(* Logix 5000 AddOnInstructionDefinition export Banner_Q5X_2000_Param_v4; software revision 33.00 *)

TYPE Banner_IOL_Port_v4 :   // UDT that has all of the data items necessary to communicate with a specific Port on a IO-Link Master
STRUCT
   Port_Controlled : INT;   // Each bit represents a port on an IO-Link Master. Set to 1 to tell AOI to control that port.
   Port_Activate : INT;   // Each bit represents a port on an IO-Link Master. When ON that port will process any commands in queue.
   Port_Read : INT;   // Each bit represents a port on an IO-Link Master. Used to determine when device AOI has requested a Read command.
   Port_Write : INT;   // Each bit represents a port on an IO-Link Master. Used to determine when device AOI has requested a Write command.
   Port_RW_Complete : INT;   // Each bit represents a port on an IO-Link Master. Tells device AOI that Read or Write request has been completed.
   Port_Device_Read : INT;
   Data_Transfer : SINT[190];   // Array to transfer data from IO-Master to device AOIs.
END_STRUCT
END_TYPE

TYPE Banner_Q5X_2000_RD_v4 :   // UDT that stores the Write Data for a Q5X.
STRUCT
   Master_Cycle_Time : INT;
   Min_Cycle_Time : INT;
   M_Sequence_Capability : INT;
   IO_Link_Version_ID : INT;
   Process_Data_Input_Length : INT;
   Process_Data_Output_Length : INT;
   Combined_Vendor_ID : DINT;   // IO-Link Vendor ID
   Vendor_ID1 : INT;
   Vendor_ID2 : INT;
   Combined_Device_ID : DINT;   // IO-Link Device ID
   Device_ID1 : INT;
   Device_ID2 : INT;
   Device_ID3 : INT;
   Serial_Number : STRING;
   Teach_State : SINT;   // 0 =IDLE, 1 = SP1 Success, 4 = Wait for Command, 5 = Busy, 7 = Error
   SP1_TP1 : SINT;   // 0 = not taught or unsuccessful, 1 = successfully taught
   SP2_TP2 : SINT;   // 0 = not taught or unsuccessful, 1 = successfully taught
   Measurement_Value : DINT;   // Measurement value in .1 mm. Dual mode the value is in percent match to taught object.
   Excess_Gain_Percent : DINT;   // Excess gain expressed as a percentage of minimum signal strength.
   Stability : INT;   // 0 = No target exists, 1 = Marginal or multiple peaks, 2 = Stable
   Multiple_Peak_State : INT;   // 0 = Multiple peaks not present, 1 = Multiple peaks present
   Emitter_Status : INT;   // 0 = Active 1 = Inactive.
   Laser_Fault_Status : INT;   // 0 = Not present, 1 Laser fault present
   BDC1_Totalizer_Counts : DINT;   // Number of totalizer edges seen on BDC1. Range: 0 to 65535.
   BDC2_Totalizer_Counts : DINT;   // Number of totalizer edges seen on BDC2. Range: 0 to 65535.
   All_Time_Run_Time : DINT;   // 0 to 2 Million. 1/4 hr increments.
   Display_String : STRING;   // String currently being displayed on the LED display of the sensor
END_STRUCT
END_TYPE

TYPE Banner_Q5X_2000_v4 :   // All of the parameters for a Q5X.
STRUCT
   Initial_Global_Read : BOOL;   // Determines if all of the IO-Link data has been read into the PLC yet
   Command : INT;   // Value placed in here will activate a read or write to a specifc IO-Link Index
   Read : Banner_Q5X_2000_RD_v4;   // Read Only Data
   Write : Banner_Q5X_2000_WD_v4;   // Write Data
   Archive_Data : Banner_Q5X_2000_WD_v4;   // Archive Write Data
   Reset : BOOL;   // Resets AOI. This will force a complete parameter read of the sensor.
END_STRUCT
END_TYPE

TYPE Banner_Q5X_2000_WD_v4 :   // UDT that stores the Write Data for a Q5X.
STRUCT
   System_Command : INT;   // See IODD file for list of commands that can be activated via the System Command interface
   Parameter_Access_Lock : SINT;   // Write access to all parameters is prohibited while value is 1. Only this parameter can be adjusted when value is 1.
   Data_Storage_Lock : SINT;   // Automatic data storage is disabled when this value is equal to 1. Read access is not affected.
   Local_Parameterization_Lock : SINT;   // Parameterization via local control elements on device is disabled.
   Local_User_Interface_Lock : SINT;   // Operation of local user interface is disabled.
   Teach_Channel : INT;   // 0 = Default, 1 = BDC1, 2 = BDC2
   BDC1_Setpoint_SP1 : DINT;   // Switch point value in .1 mm increments. Range: varies depending on sensor.
   BDC1_Setpoint_SP2 : DINT;   // In FGS mode defines second switching point parameter. Range: varies depending on sensor.
   BDC1_Swithpoint_Logic : INT;   // 0 = Light Operate, 1 = Dark Operate
   BDC1_BDC_Mode : INT;   // 1 = 1-Pt BGS, 128 = 2-Pt, 129 = Dynamic, 130 = Window or FGS, 131 = Dual
   BDC1_Hysteresis : DINT;   // Should always be 0
   BDC2_Setpoint_SP1 : DINT;   // Switch point value in .1 mm increments. Range: varies depending on sensor.
   BDC2_Setpoint_SP2 : DINT;   // In FGS mode defines second switching point parameter. Range: varies depending on sensor.
   BDC2_Switchpoint_Logic : INT;   // 0 = Light Operate, 1 = Dark Operate
   BDC2_BDC_Mode : INT;   // 1 = 1-Pt BGS, 128 = 2-Pt, 129 = Dynamic, 130 = Window or FGS, 131 = Dual
   BDC2_Hysteresis : DINT;   // Should always be 0
   Response_Speed : INT;   // 0 = 1.5 ms, 1 = 3 ms, 2 = 10 ms, 3 = 25 ms, 4 = 50 ms
   Gain : INT;   // 0 = High excess gain mode, 1 = Standard excess gain mode
   Secondary_Output_Function : INT;   // 0 = Independent Output, 1 = Complimentary Output, 2 = Remote Teach Input, 3 = Laser Off, 4 = Laser On, 5 = Master, 6 = Slave, 7 = Pulse Frequency Modulation
   Zero_Reference_Location : INT;   // 0 = Near, 1 = Far
   Shift_Zero_Reference_After_Teach : INT;   // 0 = On, 1 = Off
   Display_Read : INT;   // 0 = On, 1 = On Inverted, 2 Off, 3 Off Inverted
   Pushbutton_Lockout : INT;   // 0 = No lockout, 1 = Pushbuttons locked, 2 = Operator Lockout
   Output_Polarity : INT;   // 0 = Default, 1 = PNP, 2 = NPN.
   IOL_Filter_Time : DINT;   // Time to average IOL process data measurement between updates. Range 0 to 65535 ms.
   Include_Binary_Data : INT;   // 0 = Include, 1 = Don't Include.
   Measurement_1_Selection : INT;   // 0 = Disabled, 1 = Excess Gain, 2 = Excess Gain/10, 3 = Channel 1 Dual Mode Percent
   Measurement_2_Selection : INT;   // 0 = Disabled, 1 = Distance Measurement (divide by 10 to get cm value), 2 = Displayed Measurment, 3 = Channel 2 Dual Mode Percent
   BDC1_Delay_Mode : INT;   // 0 = Disabled, 1 = On - Off Delay, 2 = Oneshot, 3 = Totalizer
   BDC1_Delay_Timer1 : DINT;   // Time in 1 ms increments for 1.5 and 3 ms response speeds. Time in 10 ms for all other response speeds. If totalizer is selected value is in counts. Range 0 to 9999 ms.
   BDC1_Delay_Timer2 : DINT;   // Off Delay time in 1 ms increments for 1.5 and 3 ms response speeds. Time in 10 ms for all other response speeds. If totalizer is selected value is in counts. Range 0 to 9999 ms.
   BDC1_Teach_Offset_Mode : INT;   // 0 = Auto, 1 = User Selected
   BDC1_Teach_Offset : DINT;   // Teach Offset Mode must be in in User Selected for this to work. After a FGS or BGS teach the setpoint will be offset by the value stored in the parameter. Range: Values vary by sensor.
   BDC1_FGS_Window_Size : DINT;   // Teach Offset Mode must be in User Selected for this to work. Parameter sets the FGS window size. This value create a window +/- the value. Range: Values vary by sensor.
   BDC1_Auto_Thresholding : INT;   // 0 = On, 1 = Off, 2 = High Speed (Dual Mode Only)
   BDC2_Delay_Mode : INT;   // 0 = Disabled, 1 = On - Off Delay, 2 = Oneshot, 3 = Totalizer
   BDC2_Delay_Timer1 : DINT;   // Time in 1 ms increments for 1.5 and 3 ms response speeds. Time in 10 ms for all other response speeds. If totalizer is selected value is in counts. Range 0 to 9999 ms.
   BDC2_Delay_Timer2 : DINT;   // Off Delay time in 1 ms increments for 1.5 and 3 ms response speeds. Time in 10 ms for all other response speeds. If totalizer is selected value is in counts. Range 0 to 9999 ms.
   BDC2_Teach_Offset_Mode : INT;   // 0 = Auto, 1 = User Selected
   BDC2_Teach_Offset : DINT;   // Teach Offset Mode must be in in User Selected for this to work. After a FGS or BGS teach the setpoint will be offset by the value stored in the parameter. Range: Values vary by sensor.
   BDC2_FGS_Window_Size : DINT;   // Teach Offset Mode must be in User Selected for this to work. Parameter sets the FGS window size. This value create a window +/- the value. Range: Values vary by sensor.
   BDC2_Auto_Thresholding : INT;   // 0 = On, 1 = Off, 2 = High Speed (Dual Mode Only)
   Resettable_Run_Time : DINT;   // 0 to 2 Million. 1/4 hr increments.
   Near_Frequency : DINT;   // Frequency corresponding to a target at the near limit of the sensing range. Range 10 to 45000 Hz.
   Far_Frequency : DINT;   // Frequency corresponding to a target at the far limit of the sensing range. Range 10 to 45000 Hz.
   All_Time_Run_Time_Event_Time : DINT;   // 0 to 2 Million. 1/4 hr increments.
   Resettable_Run_Time_Event_Time : DINT;   // 0 to 2 Million. 1/4 hr increments.
END_STRUCT
END_TYPE

ADD_ON_INSTRUCTION Banner_Q5X_2000_Param_v4   (* revision 4.1, vendor Banner Engineering *)
// AOI to read and write parameter data to an IO-Link Q5X.
VAR_IN_OUT
   Q5X : Banner_Q5X_2000_v4; {required}
   Port_Data : Banner_IOL_Port_v4; {required}
END_VAR
VAR_INPUT
   Port : DINT; {required}
END_VAR
VAR
   Local_Control : DINT; {access None}
   Global_Read_Command_Value : INT; {access None}
   Global_Write_Command_Value : INT; {access None}
   Command_Being_Processed : BOOL; {access None}
   Update_Archive : BOOL; {access None}
   Index_Write_Inprocess : INT; {access None}
   Index_Write_Control : INT; {access None}
   Inprocess_Index : DINT; {access None}
END_VAR

ROUTINE Logic   (* ladder *)
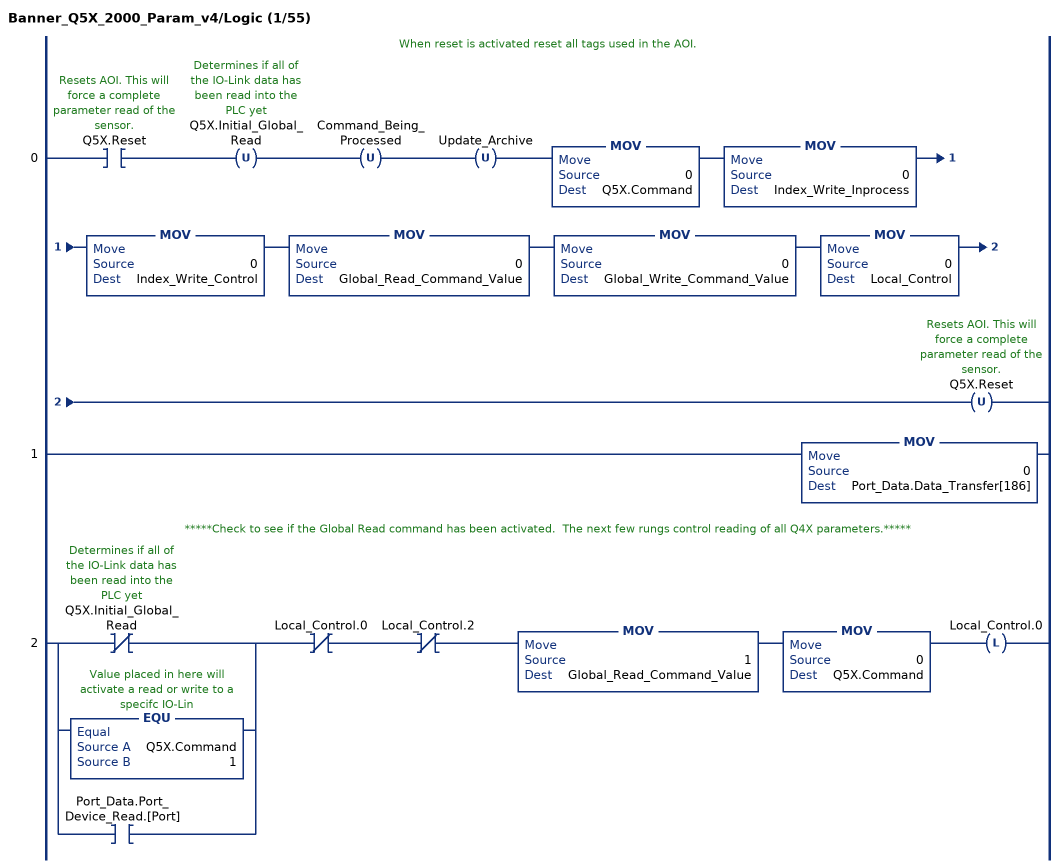
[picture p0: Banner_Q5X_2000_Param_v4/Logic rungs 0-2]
   // When reset is activated reset all tags used in the AOI.
   0: XIC(Q5X.Reset)OTU(Q5X.Initial_Global_Read)OTU(Command_Being_Processed)OTU(Update_Archive)MOV(0,Q5X.Command)MOV(0,Index_Write_Inprocess)MOV(0,Index_Write_Control)MOV(0,Global_Read_Command_Value)MOV(0,Global_Write_Command_Value)MOV(0,Local_Control)OTU(Q5X.Reset);
   1: MOV(0,Port_Data.Data_Transfer[186]);
   // *****Check to see if the Global Read command has been activated.  The next few rungs control reading of all Q4X parameters.*****
   2: [XIO(Q5X.Initial_Global_Read) ,EQU(Q5X.Command,1) ,XIC(Port_Data.Port_Device_Read.[Port]) ]XIO(Local_Control.0)XIO(Local_Control.2)MOV(1,Global_Read_Command_Value)MOV(0,Q5X.Command)OTL(Local_Control.0);
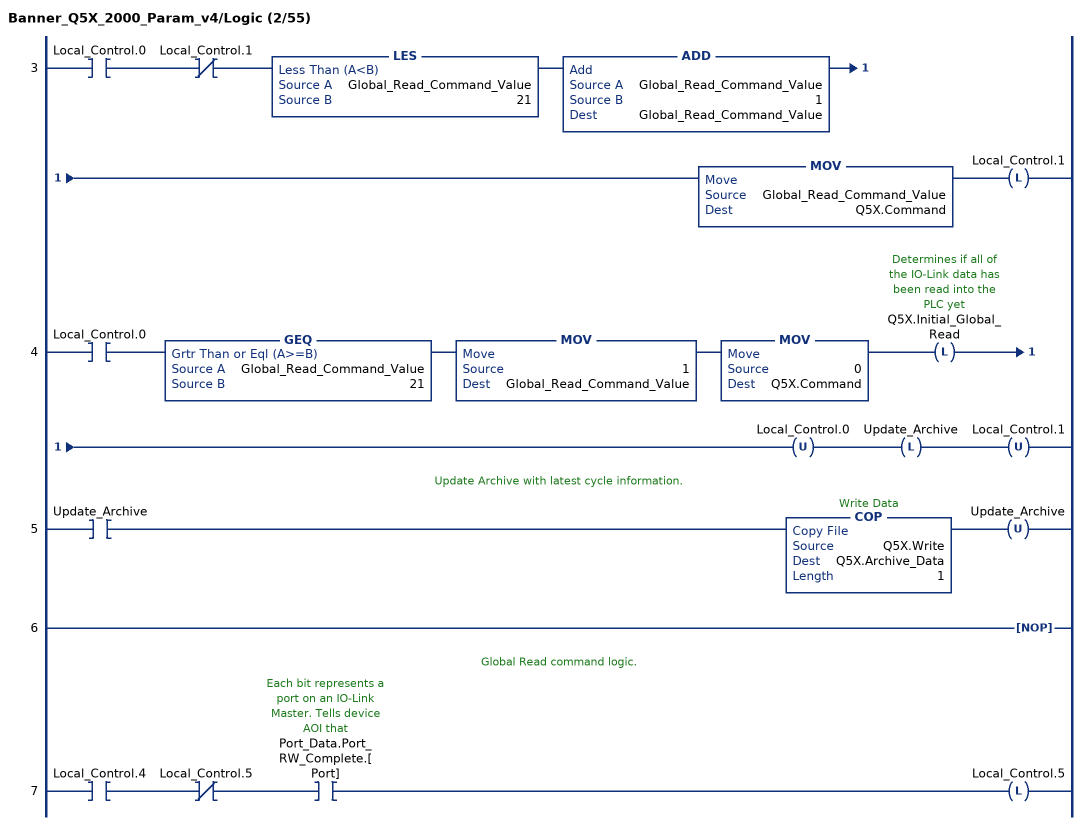
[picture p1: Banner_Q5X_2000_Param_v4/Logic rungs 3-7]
   3: XIC(Local_Control.0)XIO(Local_Control.1)LES(Global_Read_Command_Value,21)ADD(Global_Read_Command_Value,1,Global_Read_Command_Value)MOV(Global_Read_Command_Value,Q5X.Command)OTL(Local_Control.1);
   4: XIC(Local_Control.0)GEQ(Global_Read_Command_Value,21)MOV(1,Global_Read_Command_Value)MOV(0,Q5X.Command)OTL(Q5X.Initial_Global_Read)OTU(Local_Control.0)OTL(Update_Archive)OTU(Local_Control.1);
   // Update Archive with latest cycle information.
   5: XIC(Update_Archive)COP(Q5X.Write,Q5X.Archive_Data,1)OTU(Update_Archive);
   6: NOP();
   // Global Read command logic.
   7: XIC(Local_Control.4)XIO(Local_Control.5)XIC(Port_Data.Port_RW_Complete.[Port])OTL(Local_Control.5);
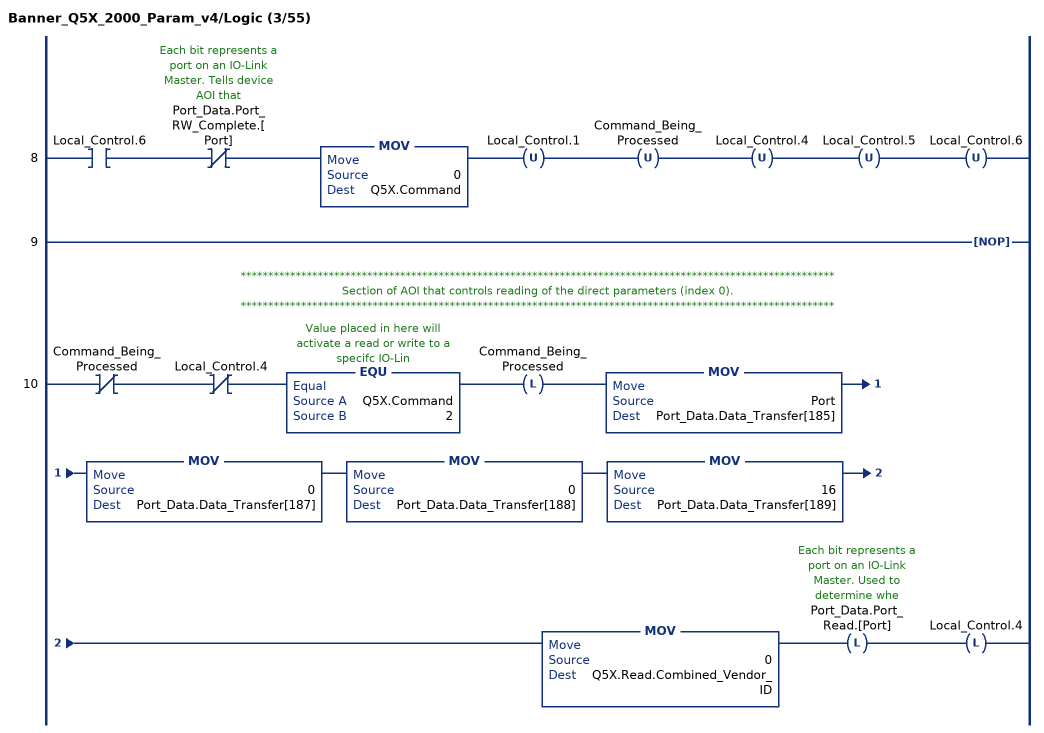
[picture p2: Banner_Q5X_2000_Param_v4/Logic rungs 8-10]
   8: XIC(Local_Control.6)XIO(Port_Data.Port_RW_Complete.[Port])MOV(0,Q5X.Command)OTU(Local_Control.1)OTU(Command_Being_Processed)OTU(Local_Control.4)OTU(Local_Control.5)OTU(Local_Control.6);
   9: NOP();
   // ************************************************************************************************************
   // Section of AOI that controls reading of the direct parameters (index 0).
   // ************************************************************************************************************
   10: XIO(Command_Being_Processed)XIO(Local_Control.4)EQU(Q5X.Command,2)OTL(Command_Being_Processed)MOV(Port,Port_Data.Data_Transfer[185])MOV(0,Port_Data.Data_Transfer[187])MOV(0,Port_Data.Data_Transfer[188])MOV(16,Port_Data.Data_Transfer[189])MOV(0,Q5X.Read.Combined_Vendor_ID)OTL(Port_Data.Port_Read.[Port])OTL(Local_Control.4);
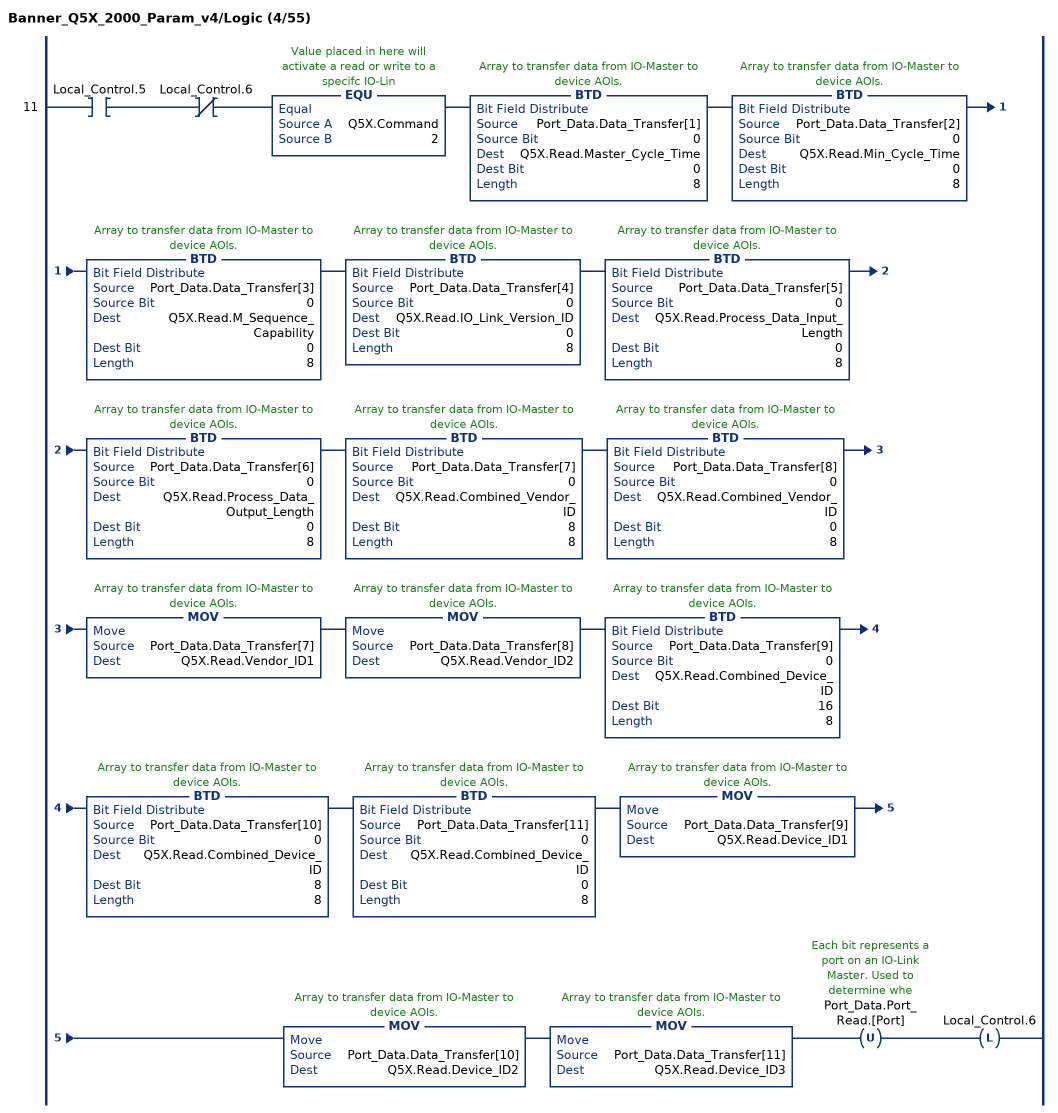
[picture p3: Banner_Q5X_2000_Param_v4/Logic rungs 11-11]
   11: XIC(Local_Control.5)XIO(Local_Control.6)EQU(Q5X.Command,2)BTD(Port_Data.Data_Transfer[1],0,Q5X.Read.Master_Cycle_Time,0,8)BTD(Port_Data.Data_Transfer[2],0,Q5X.Read.Min_Cycle_Time,0,8)BTD(Port_Data.Data_Transfer[3],0,Q5X.Read.M_Sequence_Capability,0,8)BTD(Port_Data.Data_Transfer[4],0,Q5X.Read.IO_Link_Version_ID,0,8)BTD(Port_Data.Data_Transfer[5],0,Q5X.Read.Process_Data_Input_Length,0,8)BTD(Port_Data.Data_Transfer[6],0,Q5X.Read.Process_Data_Output_Length,0,8)BTD(Port_Data.Data_Transfer[7],0,Q5X.Read.Combined_Vendor_ID,8,8)BTD(Port_Data.Data_Transfer[8],0,Q5X.Read.Combined_Vendor_ID,0,8)MOV(Port_Data.Data_Transfer[7],Q5X.Read.Vendor_ID1)MOV(Port_Data.Data_Transfer[8],Q5X.Read.Vendor_ID2)BTD(Port_Data.Data_Transfer[9],0,Q5X.Read.Combined_Device_ID,16,8)BTD(Port_Data.Data_Transfer[10],0,Q5X.Read.Combined_Device_ID,8,8)BTD(Port_Data.Data_Transfer[11],0,Q5X.Read.Combined_Device_ID,0,8)MOV(Port_Data.Data_Transfer[9],Q5X.Read.Device_ID1)MOV(Port_Data.Data_Transfer[10],Q5X.Read.Device_ID2)MOV(Port_Data.Data_Transfer[11],Q5X.Read.Device_ID3)OTU(Port_Data.Port_Read.[Port])OTL(Local_Control.6);
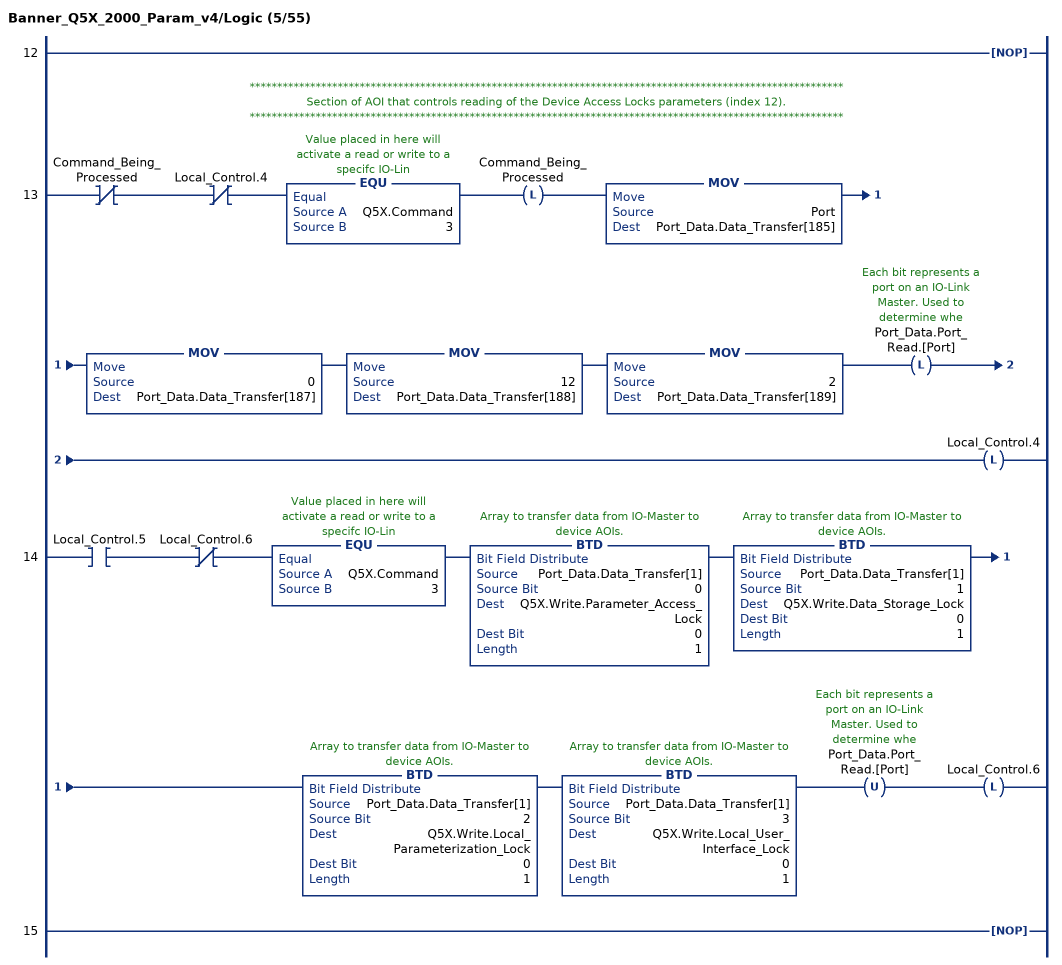
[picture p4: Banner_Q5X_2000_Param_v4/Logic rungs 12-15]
   12: NOP();
   // ************************************************************************************************************
   // Section of AOI that controls reading of the Device Access Locks parameters (index 12).
   // ************************************************************************************************************
   13: XIO(Command_Being_Processed)XIO(Local_Control.4)EQU(Q5X.Command,3)OTL(Command_Being_Processed)MOV(Port,Port_Data.Data_Transfer[185])MOV(0,Port_Data.Data_Transfer[187])MOV(12,Port_Data.Data_Transfer[188])MOV(2,Port_Data.Data_Transfer[189])OTL(Port_Data.Port_Read.[Port])OTL(Local_Control.4);
   14: XIC(Local_Control.5)XIO(Local_Control.6)EQU(Q5X.Command,3)BTD(Port_Data.Data_Transfer[1],0,Q5X.Write.Parameter_Access_Lock,0,1)BTD(Port_Data.Data_Transfer[1],1,Q5X.Write.Data_Storage_Lock,0,1)BTD(Port_Data.Data_Transfer[1],2,Q5X.Write.Local_Parameterization_Lock,0,1)BTD(Port_Data.Data_Transfer[1],3,Q5X.Write.Local_User_Interface_Lock,0,1)OTU(Port_Data.Port_Read.[Port])OTL(Local_Control.6);
   15: NOP();
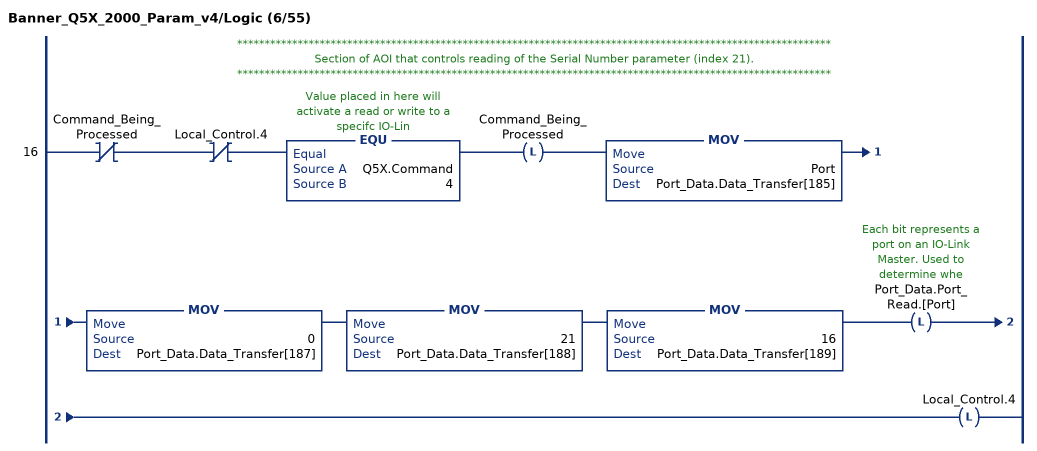
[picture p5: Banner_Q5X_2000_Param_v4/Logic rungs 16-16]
   // ************************************************************************************************************
   // Section of AOI that controls reading of the Serial Number parameter (index 21).
   // ************************************************************************************************************
   16: XIO(Command_Being_Processed)XIO(Local_Control.4)EQU(Q5X.Command,4)OTL(Command_Being_Processed)MOV(Port,Port_Data.Data_Transfer[185])MOV(0,Port_Data.Data_Transfer[187])MOV(21,Port_Data.Data_Transfer[188])MOV(16,Port_Data.Data_Transfer[189])OTL(Port_Data.Port_Read.[Port])OTL(Local_Control.4);
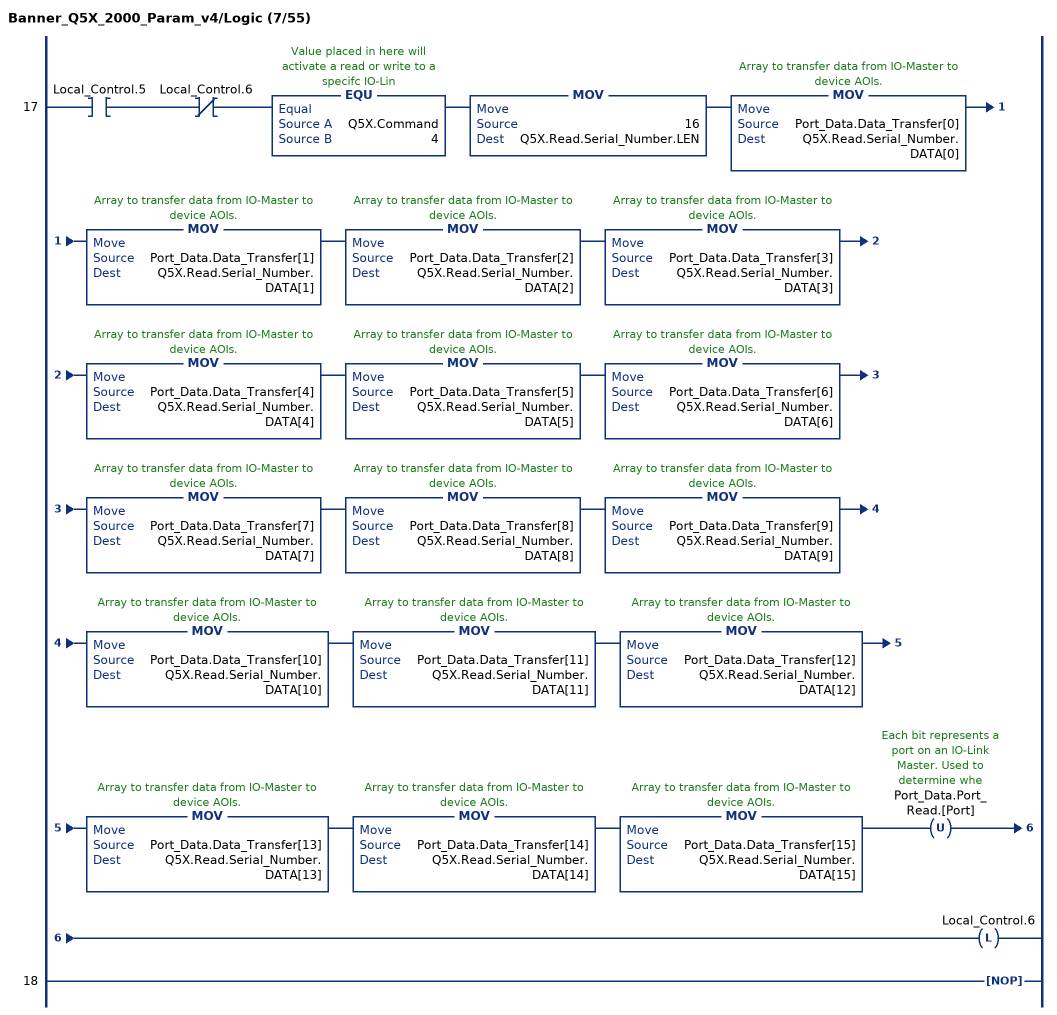
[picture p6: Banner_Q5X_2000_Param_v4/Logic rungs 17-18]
   17: XIC(Local_Control.5)XIO(Local_Control.6)EQU(Q5X.Command,4)MOV(16,Q5X.Read.Serial_Number.LEN)MOV(Port_Data.Data_Transfer[0],Q5X.Read.Serial_Number.DATA[0])MOV(Port_Data.Data_Transfer[1],Q5X.Read.Serial_Number.DATA[1])MOV(Port_Data.Data_Transfer[2],Q5X.Read.Serial_Number.DATA[2])MOV(Port_Data.Data_Transfer[3],Q5X.Read.Serial_Number.DATA[3])MOV(Port_Data.Data_Transfer[4],Q5X.Read.Serial_Number.DATA[4])MOV(Port_Data.Data_Transfer[5],Q5X.Read.Serial_Number.DATA[5])MOV(Port_Data.Data_Transfer[6],Q5X.Read.Serial_Number.DATA[6])MOV(Port_Data.Data_Transfer[7],Q5X.Read.Serial_Number.DATA[7])MOV(Port_Data.Data_Transfer[8],Q5X.Read.Serial_Number.DATA[8])MOV(Port_Data.Data_Transfer[9],Q5X.Read.Serial_Number.DATA[9])MOV(Port_Data.Data_Transfer[10],Q5X.Read.Serial_Number.DATA[10])MOV(Port_Data.Data_Transfer[11],Q5X.Read.Serial_Number.DATA[11])MOV(Port_Data.Data_Transfer[12],Q5X.Read.Serial_Number.DATA[12])MOV(Port_Data.Data_Transfer[13],Q5X.Read.Serial_Number.DATA[13])MOV(Port_Data.Data_Transfer[14],Q5X.Read.Serial_Number.DATA[14])MOV(Port_Data.Data_Transfer[15],Q5X.Read.Serial_Number.DATA[15])OTU(Port_Data.Port_Read.[Port])OTL(Local_Control.6);
   18: NOP();
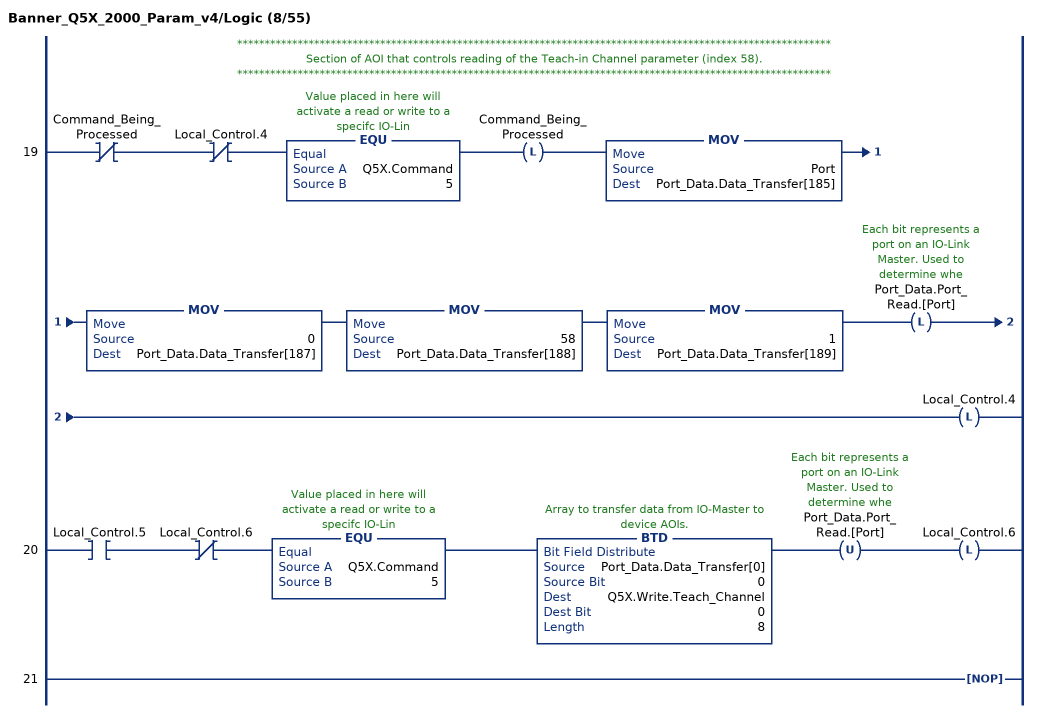
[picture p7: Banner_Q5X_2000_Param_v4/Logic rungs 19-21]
   // ************************************************************************************************************
   // Section of AOI that controls reading of the Teach-in Channel parameter (index 58).
   // ************************************************************************************************************
   19: XIO(Command_Being_Processed)XIO(Local_Control.4)EQU(Q5X.Command,5)OTL(Command_Being_Processed)MOV(Port,Port_Data.Data_Transfer[185])MOV(0,Port_Data.Data_Transfer[187])MOV(58,Port_Data.Data_Transfer[188])MOV(1,Port_Data.Data_Transfer[189])OTL(Port_Data.Port_Read.[Port])OTL(Local_Control.4);
   20: XIC(Local_Control.5)XIO(Local_Control.6)EQU(Q5X.Command,5)BTD(Port_Data.Data_Transfer[0],0,Q5X.Write.Teach_Channel,0,8)OTU(Port_Data.Port_Read.[Port])OTL(Local_Control.6);
   21: NOP();
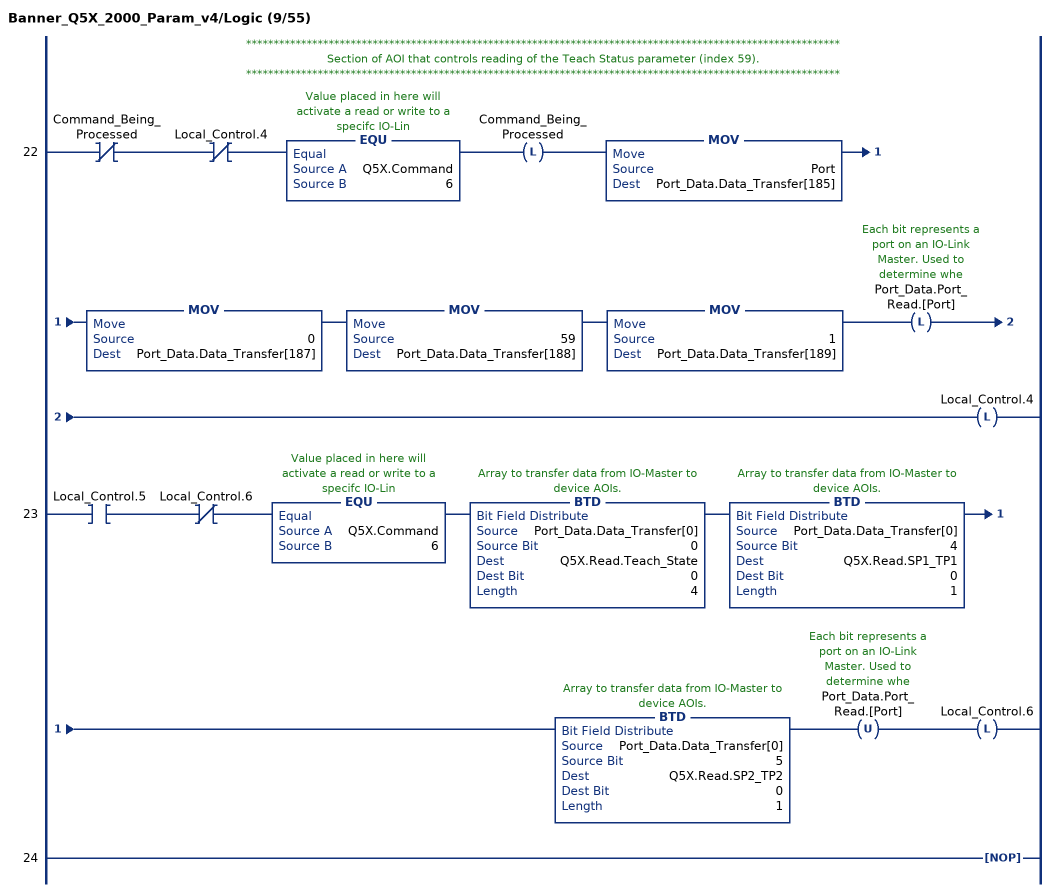
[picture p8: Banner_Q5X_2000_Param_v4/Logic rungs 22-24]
   // ************************************************************************************************************
   // Section of AOI that controls reading of the Teach Status parameter (index 59).
   // ************************************************************************************************************
   22: XIO(Command_Being_Processed)XIO(Local_Control.4)EQU(Q5X.Command,6)OTL(Command_Being_Processed)MOV(Port,Port_Data.Data_Transfer[185])MOV(0,Port_Data.Data_Transfer[187])MOV(59,Port_Data.Data_Transfer[188])MOV(1,Port_Data.Data_Transfer[189])OTL(Port_Data.Port_Read.[Port])OTL(Local_Control.4);
   23: XIC(Local_Control.5)XIO(Local_Control.6)EQU(Q5X.Command,6)BTD(Port_Data.Data_Transfer[0],0,Q5X.Read.Teach_State,0,4)BTD(Port_Data.Data_Transfer[0],4,Q5X.Read.SP1_TP1,0,1)BTD(Port_Data.Data_Transfer[0],5,Q5X.Read.SP2_TP2,0,1)OTU(Port_Data.Port_Read.[Port])OTL(Local_Control.6);
   24: NOP();
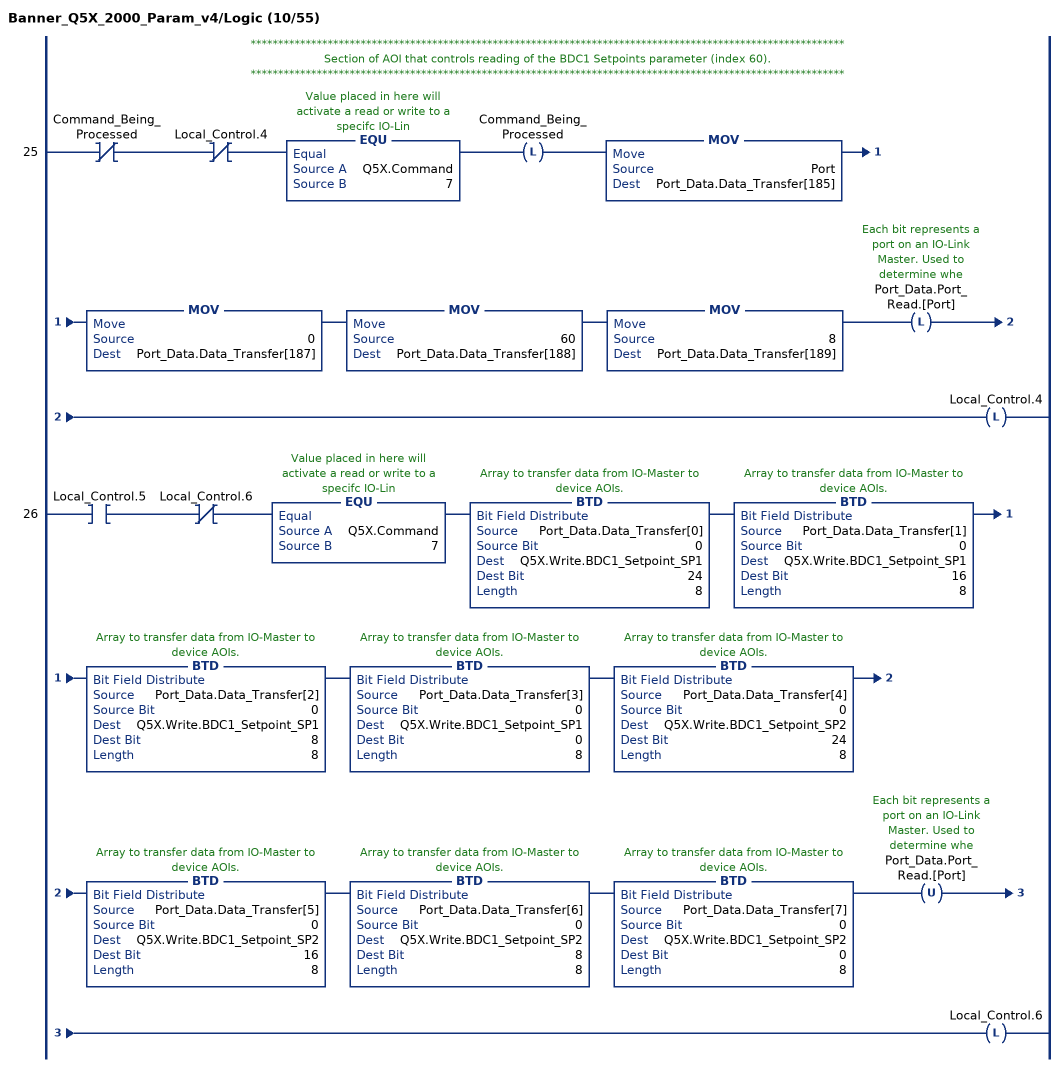
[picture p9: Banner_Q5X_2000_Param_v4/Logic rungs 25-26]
   // ************************************************************************************************************
   // Section of AOI that controls reading of the BDC1 Setpoints parameter (index 60).
   // ************************************************************************************************************
   25: XIO(Command_Being_Processed)XIO(Local_Control.4)EQU(Q5X.Command,7)OTL(Command_Being_Processed)MOV(Port,Port_Data.Data_Transfer[185])MOV(0,Port_Data.Data_Transfer[187])MOV(60,Port_Data.Data_Transfer[188])MOV(8,Port_Data.Data_Transfer[189])OTL(Port_Data.Port_Read.[Port])OTL(Local_Control.4);
   26: XIC(Local_Control.5)XIO(Local_Control.6)EQU(Q5X.Command,7)BTD(Port_Data.Data_Transfer[0],0,Q5X.Write.BDC1_Setpoint_SP1,24,8)BTD(Port_Data.Data_Transfer[1],0,Q5X.Write.BDC1_Setpoint_SP1,16,8)BTD(Port_Data.Data_Transfer[2],0,Q5X.Write.BDC1_Setpoint_SP1,8,8)BTD(Port_Data.Data_Transfer[3],0,Q5X.Write.BDC1_Setpoint_SP1,0,8)BTD(Port_Data.Data_Transfer[4],0,Q5X.Write.BDC1_Setpoint_SP2,24,8)BTD(Port_Data.Data_Transfer[5],0,Q5X.Write.BDC1_Setpoint_SP2,16,8)BTD(Port_Data.Data_Transfer[6],0,Q5X.Write.BDC1_Setpoint_SP2,8,8)BTD(Port_Data.Data_Transfer[7],0,Q5X.Write.BDC1_Setpoint_SP2,0,8)OTU(Port_Data.Port_Read.[Port])OTL(Local_Control.6);
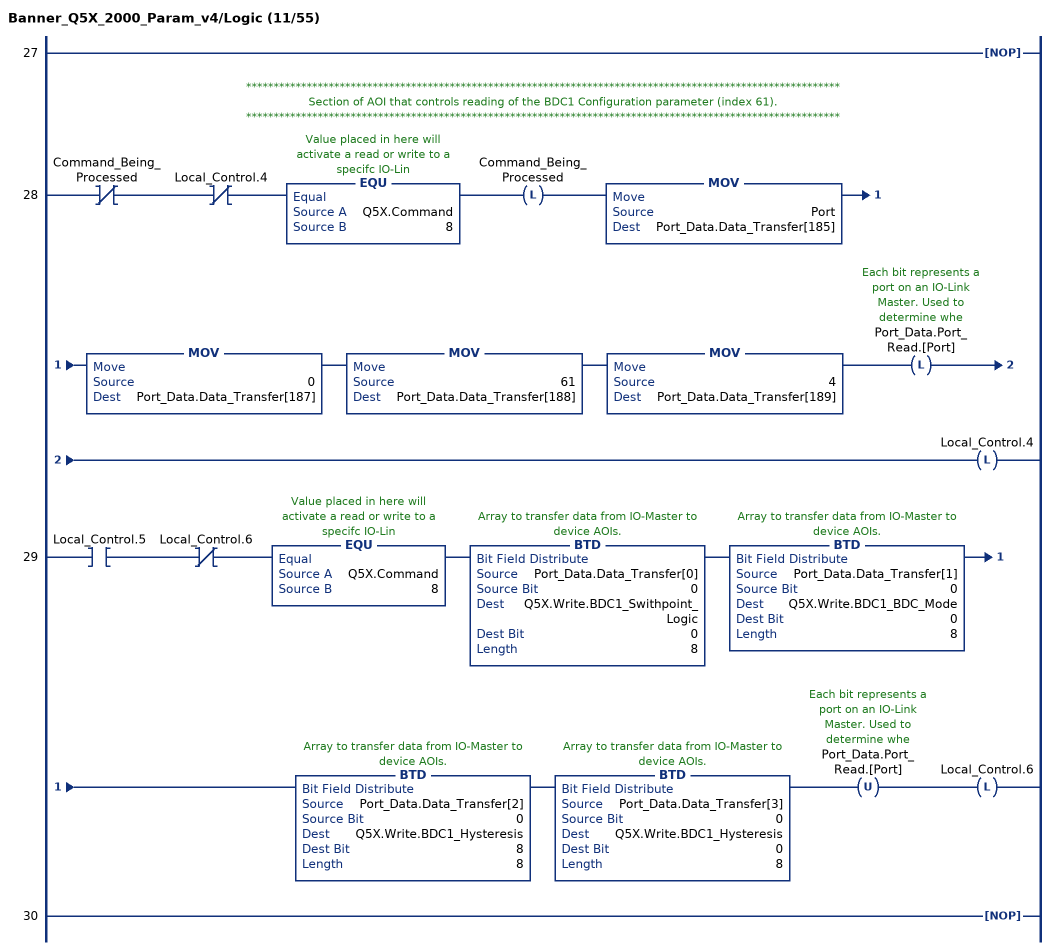
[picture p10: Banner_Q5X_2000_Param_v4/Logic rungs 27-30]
   27: NOP();
   // ************************************************************************************************************
   // Section of AOI that controls reading of the BDC1 Configuration parameter (index 61).
   // ************************************************************************************************************
   28: XIO(Command_Being_Processed)XIO(Local_Control.4)EQU(Q5X.Command,8)OTL(Command_Being_Processed)MOV(Port,Port_Data.Data_Transfer[185])MOV(0,Port_Data.Data_Transfer[187])MOV(61,Port_Data.Data_Transfer[188])MOV(4,Port_Data.Data_Transfer[189])OTL(Port_Data.Port_Read.[Port])OTL(Local_Control.4);
   29: XIC(Local_Control.5)XIO(Local_Control.6)EQU(Q5X.Command,8)BTD(Port_Data.Data_Transfer[0],0,Q5X.Write.BDC1_Swithpoint_Logic,0,8)BTD(Port_Data.Data_Transfer[1],0,Q5X.Write.BDC1_BDC_Mode,0,8)BTD(Port_Data.Data_Transfer[2],0,Q5X.Write.BDC1_Hysteresis,8,8)BTD(Port_Data.Data_Transfer[3],0,Q5X.Write.BDC1_Hysteresis,0,8)OTU(Port_Data.Port_Read.[Port])OTL(Local_Control.6);
   30: NOP();
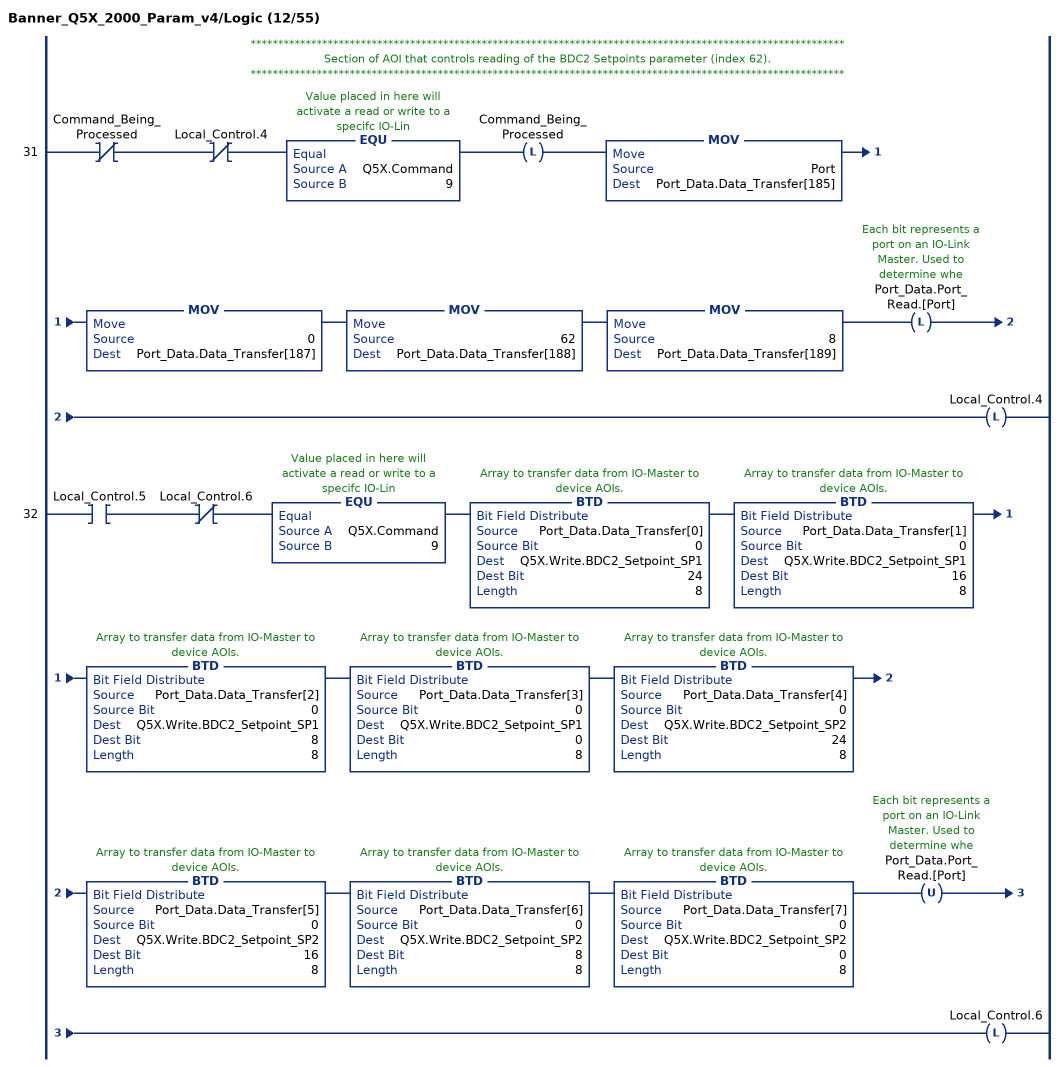
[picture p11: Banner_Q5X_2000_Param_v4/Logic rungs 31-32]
   // ************************************************************************************************************
   // Section of AOI that controls reading of the BDC2 Setpoints parameter (index 62).
   // ************************************************************************************************************
   31: XIO(Command_Being_Processed)XIO(Local_Control.4)EQU(Q5X.Command,9)OTL(Command_Being_Processed)MOV(Port,Port_Data.Data_Transfer[185])MOV(0,Port_Data.Data_Transfer[187])MOV(62,Port_Data.Data_Transfer[188])MOV(8,Port_Data.Data_Transfer[189])OTL(Port_Data.Port_Read.[Port])OTL(Local_Control.4);
   32: XIC(Local_Control.5)XIO(Local_Control.6)EQU(Q5X.Command,9)BTD(Port_Data.Data_Transfer[0],0,Q5X.Write.BDC2_Setpoint_SP1,24,8)BTD(Port_Data.Data_Transfer[1],0,Q5X.Write.BDC2_Setpoint_SP1,16,8)BTD(Port_Data.Data_Transfer[2],0,Q5X.Write.BDC2_Setpoint_SP1,8,8)BTD(Port_Data.Data_Transfer[3],0,Q5X.Write.BDC2_Setpoint_SP1,0,8)BTD(Port_Data.Data_Transfer[4],0,Q5X.Write.BDC2_Setpoint_SP2,24,8)BTD(Port_Data.Data_Transfer[5],0,Q5X.Write.BDC2_Setpoint_SP2,16,8)BTD(Port_Data.Data_Transfer[6],0,Q5X.Write.BDC2_Setpoint_SP2,8,8)BTD(Port_Data.Data_Transfer[7],0,Q5X.Write.BDC2_Setpoint_SP2,0,8)OTU(Port_Data.Port_Read.[Port])OTL(Local_Control.6);
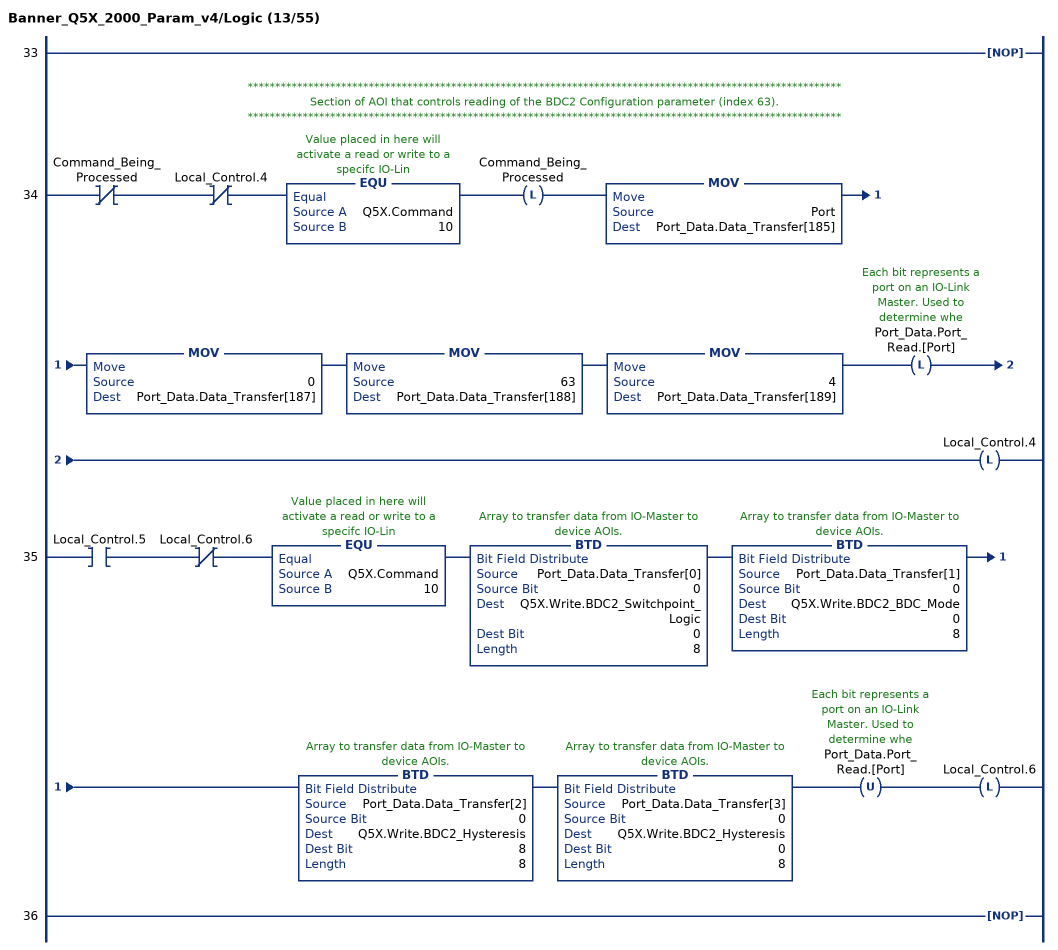
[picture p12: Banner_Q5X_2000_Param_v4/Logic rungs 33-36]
   33: NOP();
   // ************************************************************************************************************
   // Section of AOI that controls reading of the BDC2 Configuration parameter (index 63).
   // ************************************************************************************************************
   34: XIO(Command_Being_Processed)XIO(Local_Control.4)EQU(Q5X.Command,10)OTL(Command_Being_Processed)MOV(Port,Port_Data.Data_Transfer[185])MOV(0,Port_Data.Data_Transfer[187])MOV(63,Port_Data.Data_Transfer[188])MOV(4,Port_Data.Data_Transfer[189])OTL(Port_Data.Port_Read.[Port])OTL(Local_Control.4);
   35: XIC(Local_Control.5)XIO(Local_Control.6)EQU(Q5X.Command,10)BTD(Port_Data.Data_Transfer[0],0,Q5X.Write.BDC2_Switchpoint_Logic,0,8)BTD(Port_Data.Data_Transfer[1],0,Q5X.Write.BDC2_BDC_Mode,0,8)BTD(Port_Data.Data_Transfer[2],0,Q5X.Write.BDC2_Hysteresis,8,8)BTD(Port_Data.Data_Transfer[3],0,Q5X.Write.BDC2_Hysteresis,0,8)OTU(Port_Data.Port_Read.[Port])OTL(Local_Control.6);
   36: NOP();
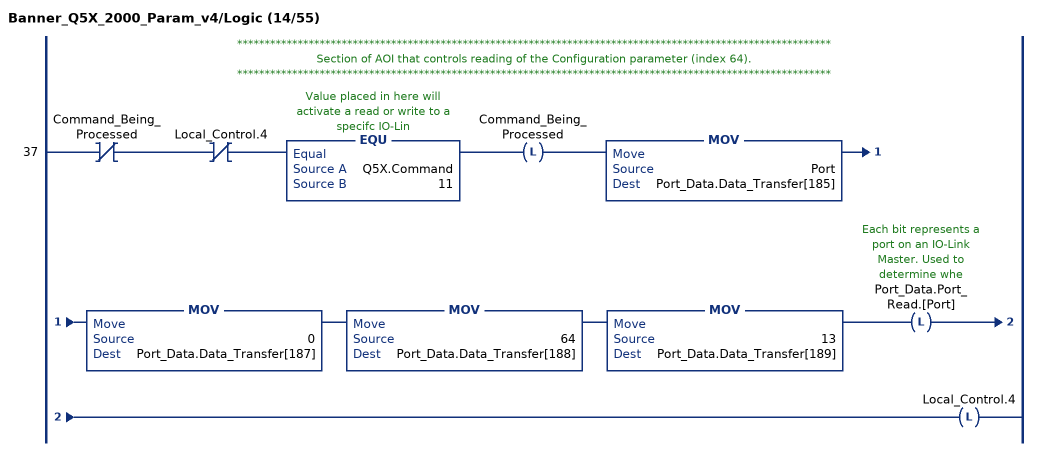
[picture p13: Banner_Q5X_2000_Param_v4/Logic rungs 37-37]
   // ************************************************************************************************************
   // Section of AOI that controls reading of the Configuration parameter (index 64).
   // ************************************************************************************************************
   37: XIO(Command_Being_Processed)XIO(Local_Control.4)EQU(Q5X.Command,11)OTL(Command_Being_Processed)MOV(Port,Port_Data.Data_Transfer[185])MOV(0,Port_Data.Data_Transfer[187])MOV(64,Port_Data.Data_Transfer[188])MOV(13,Port_Data.Data_Transfer[189])OTL(Port_Data.Port_Read.[Port])OTL(Local_Control.4);
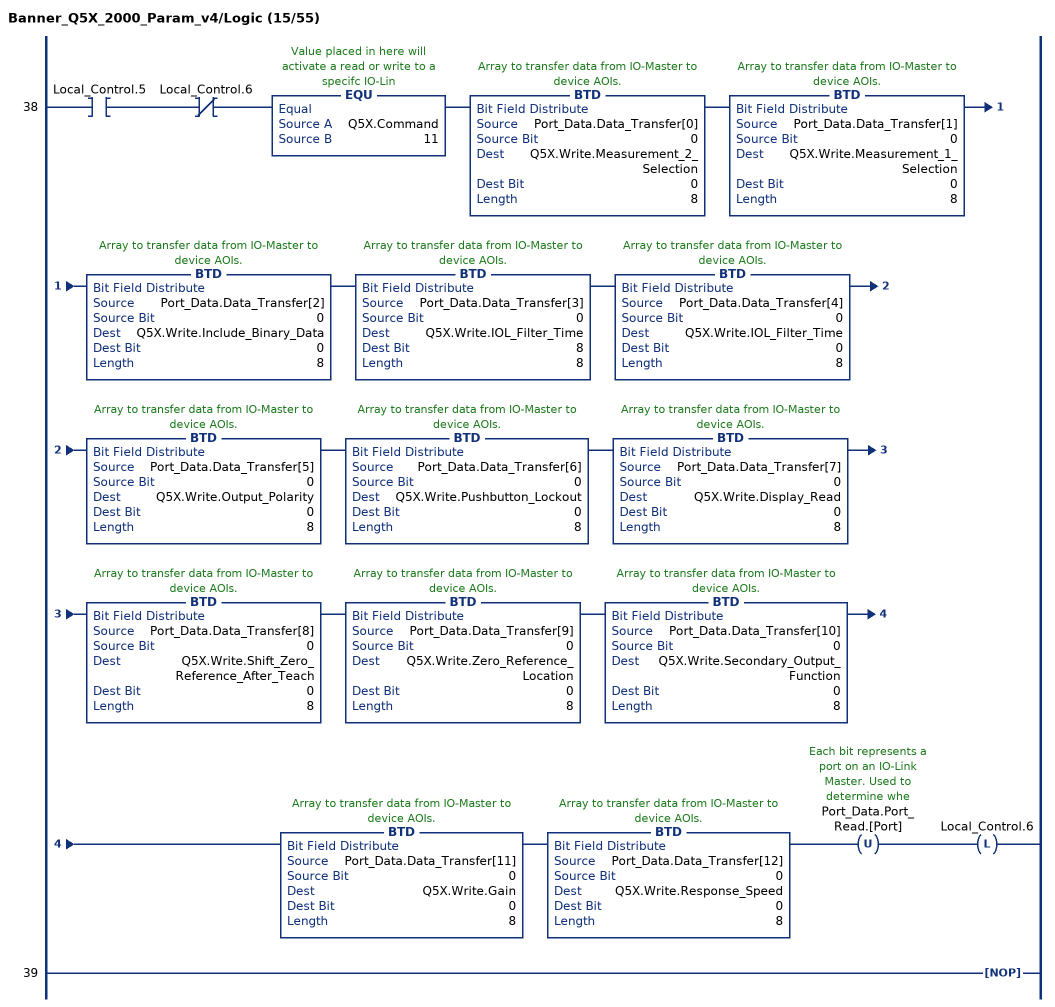
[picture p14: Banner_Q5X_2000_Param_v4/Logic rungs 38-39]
   38: XIC(Local_Control.5)XIO(Local_Control.6)EQU(Q5X.Command,11)BTD(Port_Data.Data_Transfer[0],0,Q5X.Write.Measurement_2_Selection,0,8)BTD(Port_Data.Data_Transfer[1],0,Q5X.Write.Measurement_1_Selection,0,8)BTD(Port_Data.Data_Transfer[2],0,Q5X.Write.Include_Binary_Data,0,8)BTD(Port_Data.Data_Transfer[3],0,Q5X.Write.IOL_Filter_Time,8,8)BTD(Port_Data.Data_Transfer[4],0,Q5X.Write.IOL_Filter_Time,0,8)BTD(Port_Data.Data_Transfer[5],0,Q5X.Write.Output_Polarity,0,8)BTD(Port_Data.Data_Transfer[6],0,Q5X.Write.Pushbutton_Lockout,0,8)BTD(Port_Data.Data_Transfer[7],0,Q5X.Write.Display_Read,0,8)BTD(Port_Data.Data_Transfer[8],0,Q5X.Write.Shift_Zero_Reference_After_Teach,0,8)BTD(Port_Data.Data_Transfer[9],0,Q5X.Write.Zero_Reference_Location,0,8)BTD(Port_Data.Data_Transfer[10],0,Q5X.Write.Secondary_Output_Function,0,8)BTD(Port_Data.Data_Transfer[11],0,Q5X.Write.Gain,0,8)BTD(Port_Data.Data_Transfer[12],0,Q5X.Write.Response_Speed,0,8)OTU(Port_Data.Port_Read.[Port])OTL(Local_Control.6);
   39: NOP();
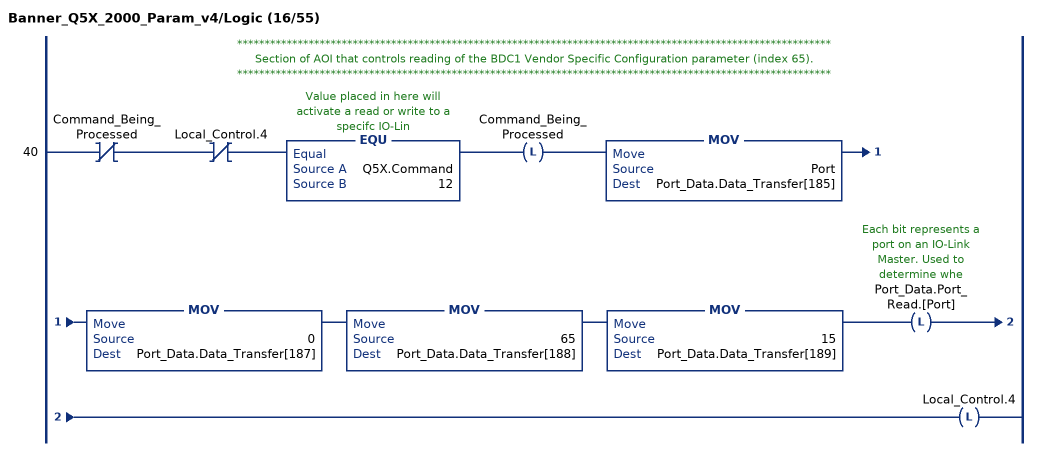
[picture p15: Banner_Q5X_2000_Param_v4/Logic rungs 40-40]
   // ************************************************************************************************************
   // Section of AOI that controls reading of the BDC1 Vendor Specific Configuration parameter (index 65).
   // ************************************************************************************************************
   40: XIO(Command_Being_Processed)XIO(Local_Control.4)EQU(Q5X.Command,12)OTL(Command_Being_Processed)MOV(Port,Port_Data.Data_Transfer[185])MOV(0,Port_Data.Data_Transfer[187])MOV(65,Port_Data.Data_Transfer[188])MOV(15,Port_Data.Data_Transfer[189])OTL(Port_Data.Port_Read.[Port])OTL(Local_Control.4);
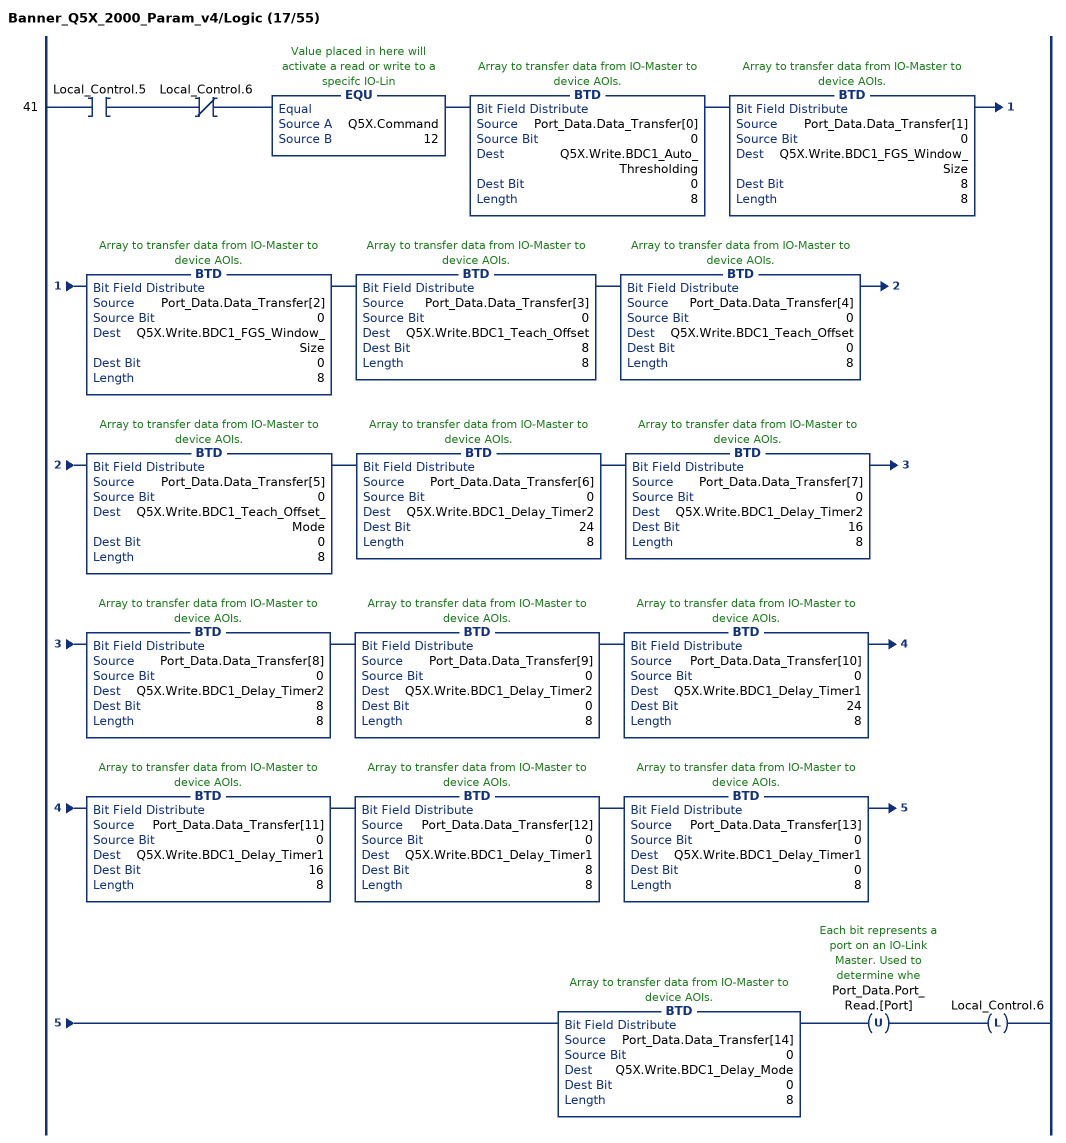
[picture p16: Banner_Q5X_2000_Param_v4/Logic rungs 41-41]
   41: XIC(Local_Control.5)XIO(Local_Control.6)EQU(Q5X.Command,12)BTD(Port_Data.Data_Transfer[0],0,Q5X.Write.BDC1_Auto_Thresholding,0,8)BTD(Port_Data.Data_Transfer[1],0,Q5X.Write.BDC1_FGS_Window_Size,8,8)BTD(Port_Data.Data_Transfer[2],0,Q5X.Write.BDC1_FGS_Window_Size,0,8)BTD(Port_Data.Data_Transfer[3],0,Q5X.Write.BDC1_Teach_Offset,8,8)BTD(Port_Data.Data_Transfer[4],0,Q5X.Write.BDC1_Teach_Offset,0,8)BTD(Port_Data.Data_Transfer[5],0,Q5X.Write.BDC1_Teach_Offset_Mode,0,8)BTD(Port_Data.Data_Transfer[6],0,Q5X.Write.BDC1_Delay_Timer2,24,8)BTD(Port_Data.Data_Transfer[7],0,Q5X.Write.BDC1_Delay_Timer2,16,8)BTD(Port_Data.Data_Transfer[8],0,Q5X.Write.BDC1_Delay_Timer2,8,8)BTD(Port_Data.Data_Transfer[9],0,Q5X.Write.BDC1_Delay_Timer2,0,8)BTD(Port_Data.Data_Transfer[10],0,Q5X.Write.BDC1_Delay_Timer1,24,8)BTD(Port_Data.Data_Transfer[11],0,Q5X.Write.BDC1_Delay_Timer1,16,8)BTD(Port_Data.Data_Transfer[12],0,Q5X.Write.BDC1_Delay_Timer1,8,8)BTD(Port_Data.Data_Transfer[13],0,Q5X.Write.BDC1_Delay_Timer1,0,8)BTD(Port_Data.Data_Transfer[14],0,Q5X.Write.BDC1_Delay_Mode,0,8)OTU(Port_Data.Port_Read.[Port])OTL(Local_Control.6);
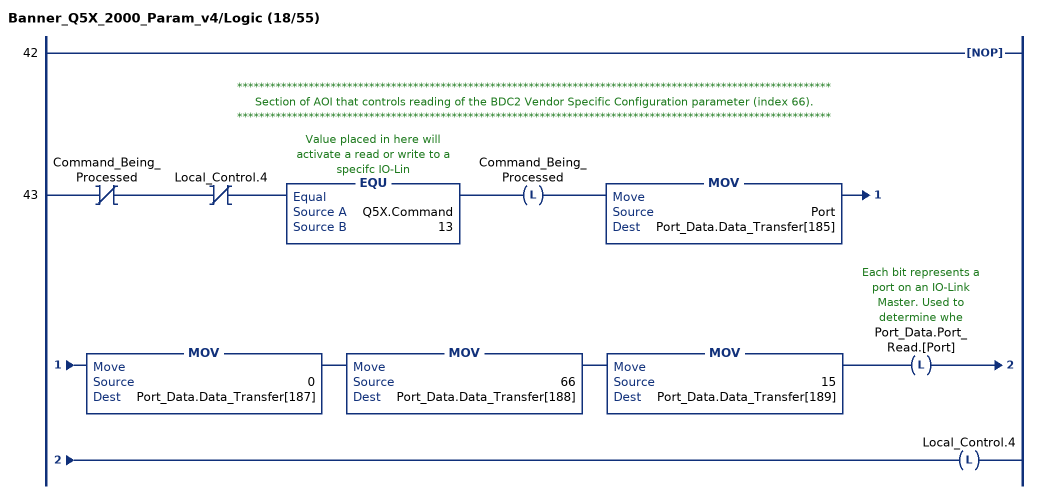
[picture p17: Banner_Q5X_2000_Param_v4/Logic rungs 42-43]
   42: NOP();
   // ************************************************************************************************************
   // Section of AOI that controls reading of the BDC2 Vendor Specific Configuration parameter (index 66).
   // ************************************************************************************************************
   43: XIO(Command_Being_Processed)XIO(Local_Control.4)EQU(Q5X.Command,13)OTL(Command_Being_Processed)MOV(Port,Port_Data.Data_Transfer[185])MOV(0,Port_Data.Data_Transfer[187])MOV(66,Port_Data.Data_Transfer[188])MOV(15,Port_Data.Data_Transfer[189])OTL(Port_Data.Port_Read.[Port])OTL(Local_Control.4);
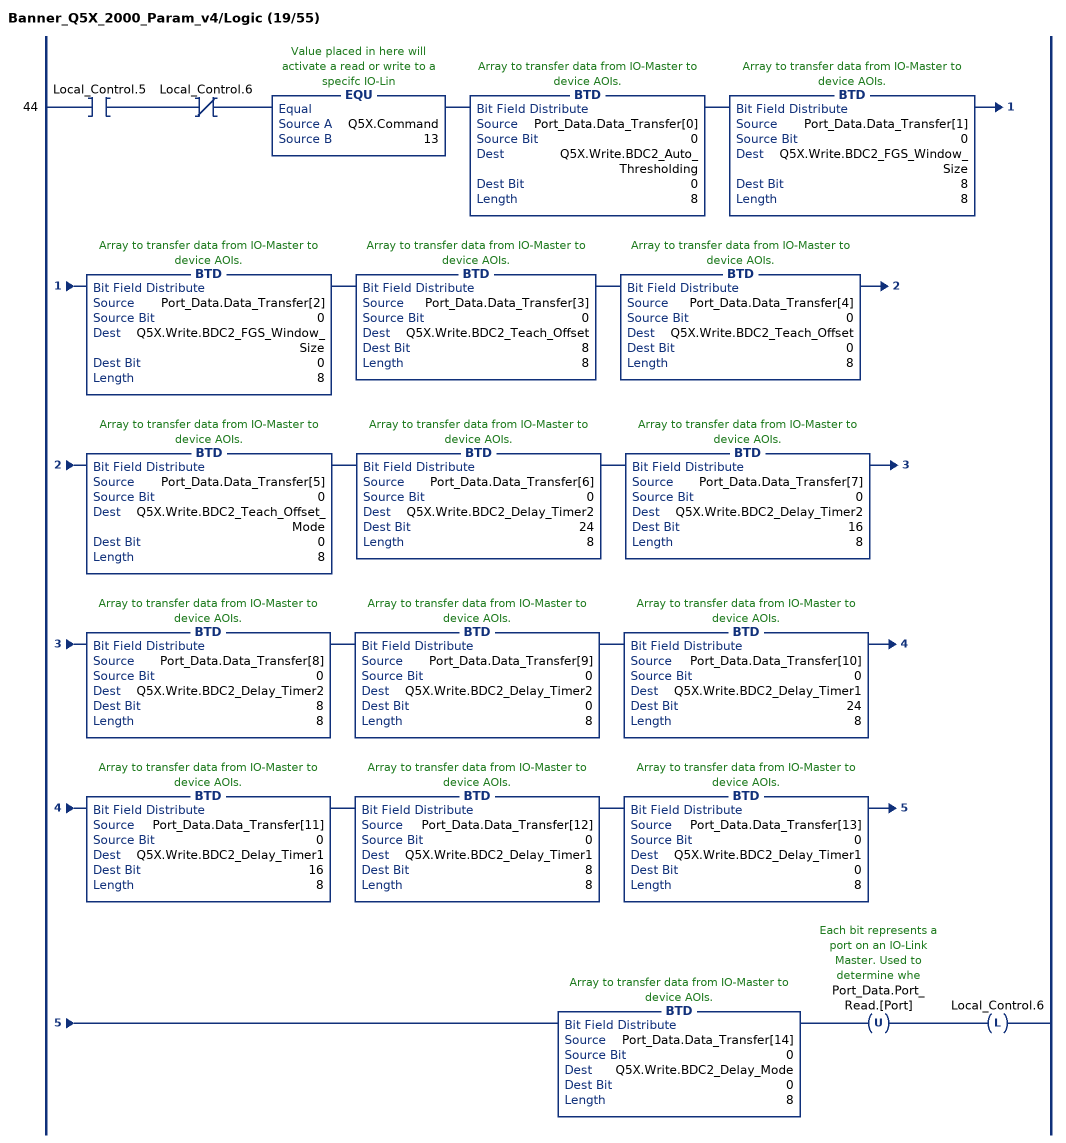
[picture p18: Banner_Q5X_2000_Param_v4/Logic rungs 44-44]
   44: XIC(Local_Control.5)XIO(Local_Control.6)EQU(Q5X.Command,13)BTD(Port_Data.Data_Transfer[0],0,Q5X.Write.BDC2_Auto_Thresholding,0,8)BTD(Port_Data.Data_Transfer[1],0,Q5X.Write.BDC2_FGS_Window_Size,8,8)BTD(Port_Data.Data_Transfer[2],0,Q5X.Write.BDC2_FGS_Window_Size,0,8)BTD(Port_Data.Data_Transfer[3],0,Q5X.Write.BDC2_Teach_Offset,8,8)BTD(Port_Data.Data_Transfer[4],0,Q5X.Write.BDC2_Teach_Offset,0,8)BTD(Port_Data.Data_Transfer[5],0,Q5X.Write.BDC2_Teach_Offset_Mode,0,8)BTD(Port_Data.Data_Transfer[6],0,Q5X.Write.BDC2_Delay_Timer2,24,8)BTD(Port_Data.Data_Transfer[7],0,Q5X.Write.BDC2_Delay_Timer2,16,8)BTD(Port_Data.Data_Transfer[8],0,Q5X.Write.BDC2_Delay_Timer2,8,8)BTD(Port_Data.Data_Transfer[9],0,Q5X.Write.BDC2_Delay_Timer2,0,8)BTD(Port_Data.Data_Transfer[10],0,Q5X.Write.BDC2_Delay_Timer1,24,8)BTD(Port_Data.Data_Transfer[11],0,Q5X.Write.BDC2_Delay_Timer1,16,8)BTD(Port_Data.Data_Transfer[12],0,Q5X.Write.BDC2_Delay_Timer1,8,8)BTD(Port_Data.Data_Transfer[13],0,Q5X.Write.BDC2_Delay_Timer1,0,8)BTD(Port_Data.Data_Transfer[14],0,Q5X.Write.BDC2_Delay_Mode,0,8)OTU(Port_Data.Port_Read.[Port])OTL(Local_Control.6);
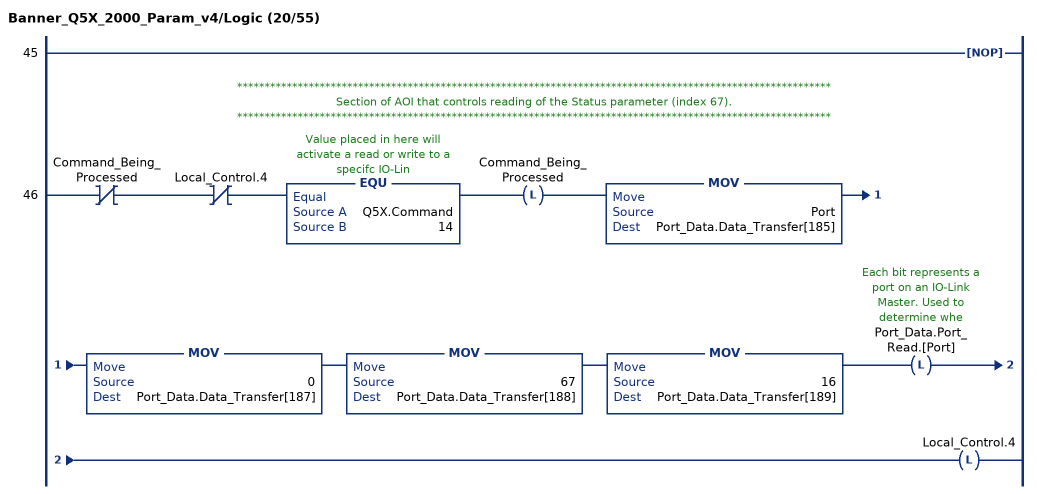
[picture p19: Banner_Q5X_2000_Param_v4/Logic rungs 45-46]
   45: NOP();
   // ************************************************************************************************************
   // Section of AOI that controls reading of the Status parameter (index 67).
   // ************************************************************************************************************
   46: XIO(Command_Being_Processed)XIO(Local_Control.4)EQU(Q5X.Command,14)OTL(Command_Being_Processed)MOV(Port,Port_Data.Data_Transfer[185])MOV(0,Port_Data.Data_Transfer[187])MOV(67,Port_Data.Data_Transfer[188])MOV(16,Port_Data.Data_Transfer[189])OTL(Port_Data.Port_Read.[Port])OTL(Local_Control.4);
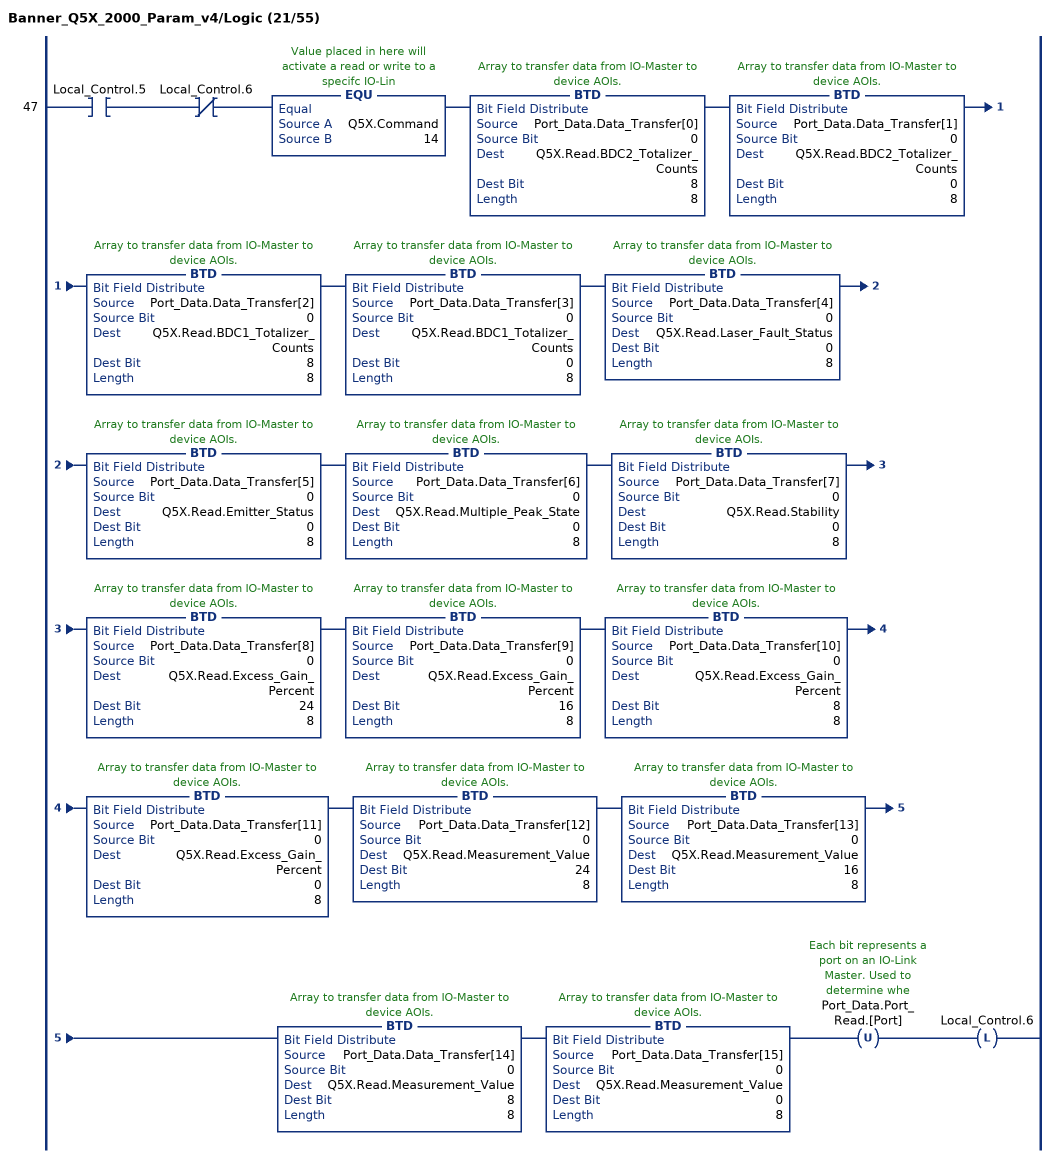
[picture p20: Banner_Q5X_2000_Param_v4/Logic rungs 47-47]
   47: XIC(Local_Control.5)XIO(Local_Control.6)EQU(Q5X.Command,14)BTD(Port_Data.Data_Transfer[0],0,Q5X.Read.BDC2_Totalizer_Counts,8,8)BTD(Port_Data.Data_Transfer[1],0,Q5X.Read.BDC2_Totalizer_Counts,0,8)BTD(Port_Data.Data_Transfer[2],0,Q5X.Read.BDC1_Totalizer_Counts,8,8)BTD(Port_Data.Data_Transfer[3],0,Q5X.Read.BDC1_Totalizer_Counts,0,8)BTD(Port_Data.Data_Transfer[4],0,Q5X.Read.Laser_Fault_Status,0,8)BTD(Port_Data.Data_Transfer[5],0,Q5X.Read.Emitter_Status,0,8)BTD(Port_Data.Data_Transfer[6],0,Q5X.Read.Multiple_Peak_State,0,8)BTD(Port_Data.Data_Transfer[7],0,Q5X.Read.Stability,0,8)BTD(Port_Data.Data_Transfer[8],0,Q5X.Read.Excess_Gain_Percent,24,8)BTD(Port_Data.Data_Transfer[9],0,Q5X.Read.Excess_Gain_Percent,16,8)BTD(Port_Data.Data_Transfer[10],0,Q5X.Read.Excess_Gain_Percent,8,8)BTD(Port_Data.Data_Transfer[11],0,Q5X.Read.Excess_Gain_Percent,0,8)BTD(Port_Data.Data_Transfer[12],0,Q5X.Read.Measurement_Value,24,8)BTD(Port_Data.Data_Transfer[13],0,Q5X.Read.Measurement_Value,16,8)BTD(Port_Data.Data_Transfer[14],0,Q5X.Read.Measurement_Value,8,8)BTD(Port_Data.Data_Transfer[15],0,Q5X.Read.Measurement_Value,0,8)OTU(Port_Data.Port_Read.[Port])OTL(Local_Control.6);
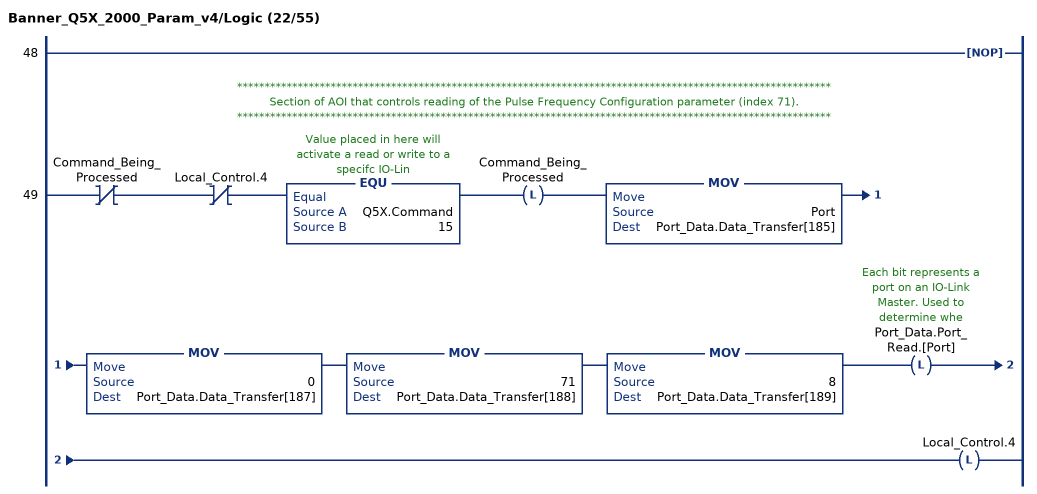
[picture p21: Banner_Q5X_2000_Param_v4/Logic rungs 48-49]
   48: NOP();
   // ************************************************************************************************************
   // Section of AOI that controls reading of the Pulse Frequency Configuration parameter (index 71).
   // ************************************************************************************************************
   49: XIO(Command_Being_Processed)XIO(Local_Control.4)EQU(Q5X.Command,15)OTL(Command_Being_Processed)MOV(Port,Port_Data.Data_Transfer[185])MOV(0,Port_Data.Data_Transfer[187])MOV(71,Port_Data.Data_Transfer[188])MOV(8,Port_Data.Data_Transfer[189])OTL(Port_Data.Port_Read.[Port])OTL(Local_Control.4);
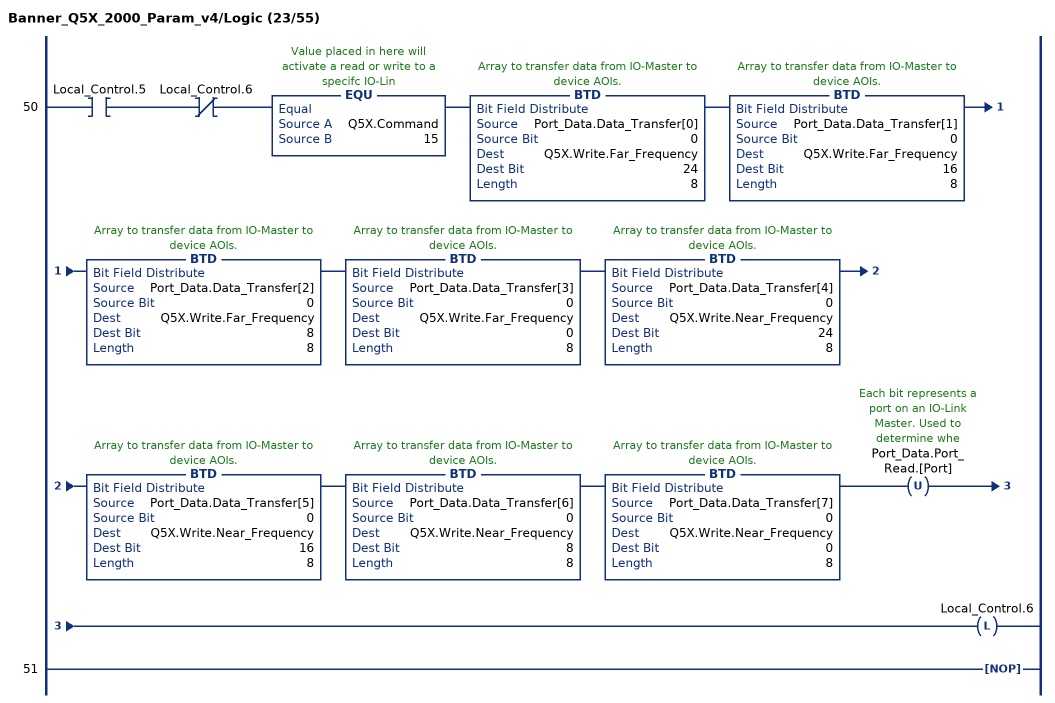
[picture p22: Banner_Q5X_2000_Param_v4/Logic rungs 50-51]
   50: XIC(Local_Control.5)XIO(Local_Control.6)EQU(Q5X.Command,15)BTD(Port_Data.Data_Transfer[0],0,Q5X.Write.Far_Frequency,24,8)BTD(Port_Data.Data_Transfer[1],0,Q5X.Write.Far_Frequency,16,8)BTD(Port_Data.Data_Transfer[2],0,Q5X.Write.Far_Frequency,8,8)BTD(Port_Data.Data_Transfer[3],0,Q5X.Write.Far_Frequency,0,8)BTD(Port_Data.Data_Transfer[4],0,Q5X.Write.Near_Frequency,24,8)BTD(Port_Data.Data_Transfer[5],0,Q5X.Write.Near_Frequency,16,8)BTD(Port_Data.Data_Transfer[6],0,Q5X.Write.Near_Frequency,8,8)BTD(Port_Data.Data_Transfer[7],0,Q5X.Write.Near_Frequency,0,8)OTU(Port_Data.Port_Read.[Port])OTL(Local_Control.6);
   51: NOP();
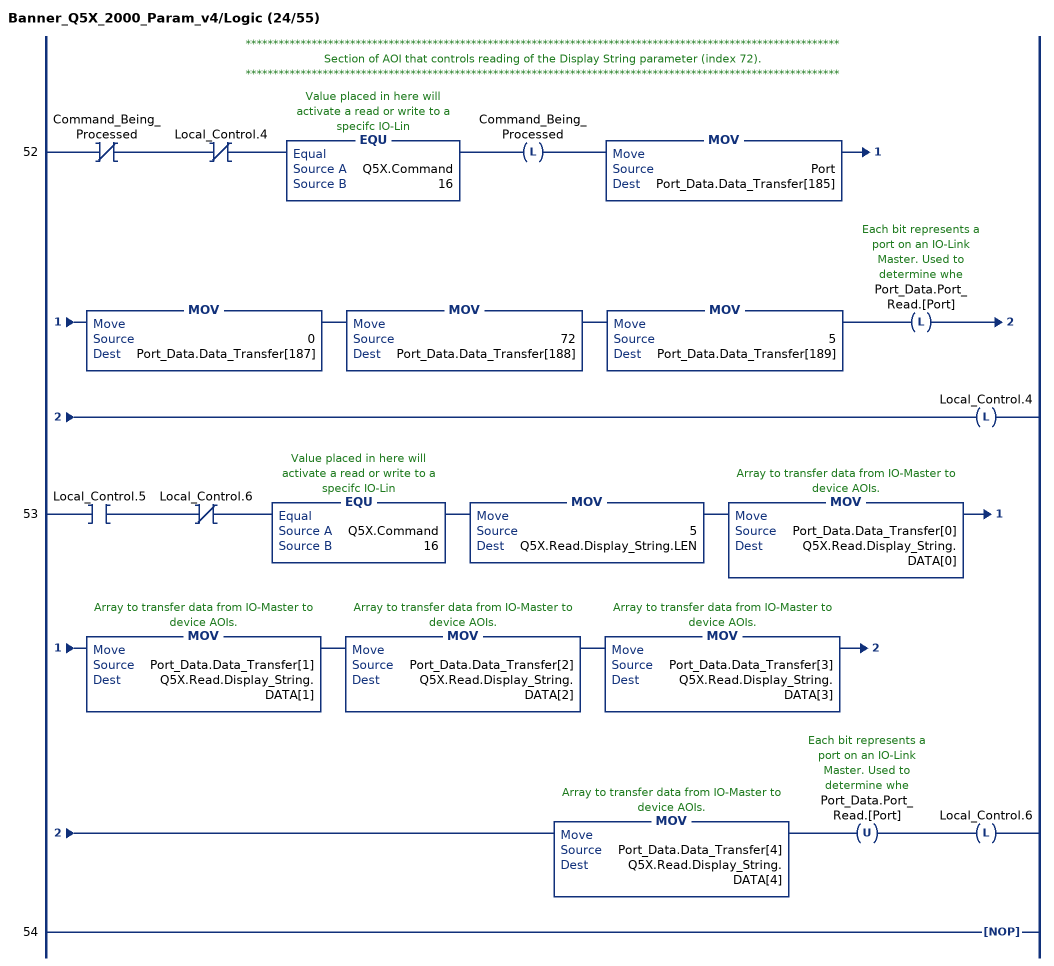
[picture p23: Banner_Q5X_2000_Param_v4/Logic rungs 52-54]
   // ************************************************************************************************************
   // Section of AOI that controls reading of the Display String parameter (index 72).
   // ************************************************************************************************************
   52: XIO(Command_Being_Processed)XIO(Local_Control.4)EQU(Q5X.Command,16)OTL(Command_Being_Processed)MOV(Port,Port_Data.Data_Transfer[185])MOV(0,Port_Data.Data_Transfer[187])MOV(72,Port_Data.Data_Transfer[188])MOV(5,Port_Data.Data_Transfer[189])OTL(Port_Data.Port_Read.[Port])OTL(Local_Control.4);
   53: XIC(Local_Control.5)XIO(Local_Control.6)EQU(Q5X.Command,16)MOV(5,Q5X.Read.Display_String.LEN)MOV(Port_Data.Data_Transfer[0],Q5X.Read.Display_String.DATA[0])MOV(Port_Data.Data_Transfer[1],Q5X.Read.Display_String.DATA[1])MOV(Port_Data.Data_Transfer[2],Q5X.Read.Display_String.DATA[2])MOV(Port_Data.Data_Transfer[3],Q5X.Read.Display_String.DATA[3])MOV(Port_Data.Data_Transfer[4],Q5X.Read.Display_String.DATA[4])OTU(Port_Data.Port_Read.[Port])OTL(Local_Control.6);
   54: NOP();
